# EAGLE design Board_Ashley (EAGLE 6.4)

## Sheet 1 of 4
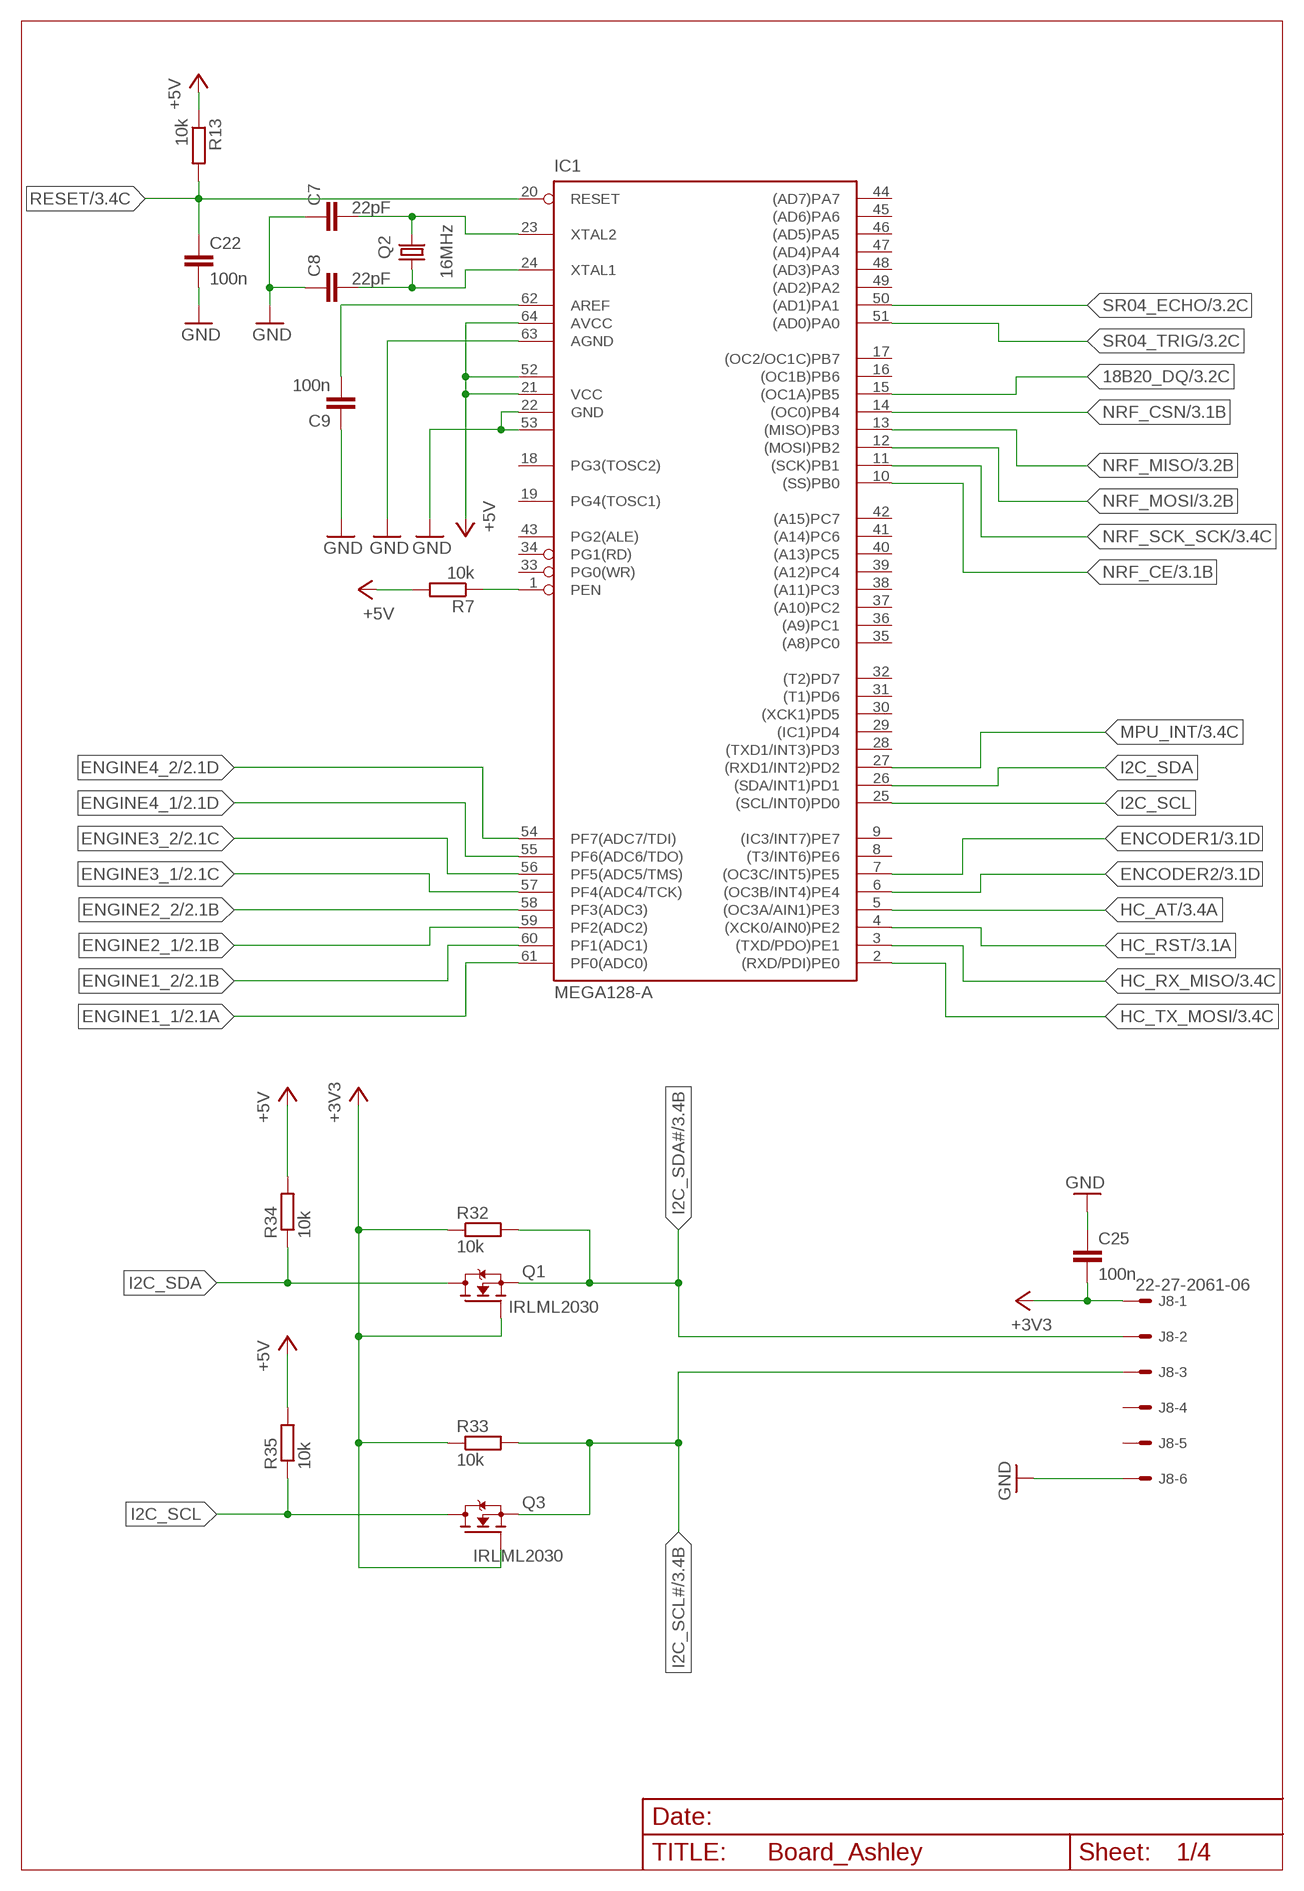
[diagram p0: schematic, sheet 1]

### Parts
C7  22pF  C-EUC0805  [C0805]
C8  22pF  C-EUC0805  [C0805]
C9  100n  C-EUC0805  [C0805]
C22  100n  C-EUC0805  [C0805]
C25  100n  C-EUC0805  [C0805]
IC1  MEGA128-A  [TQFP64]
J8  22-27-2061-06  [6410-06]
Q1  IRLML2030  [SOT23]
Q2  16MHz  CRYSTALHC49U-V  [HC49U-V]
Q3  IRLML2030  [SOT23]
R7  10k  R-EU_R0805  [R0805]
R13  10k  R-EU_R0805  [R0805]
R32  10k  R-EU_R0805  [R0805]
R33  10k  R-EU_R0805  [R0805]
R34  10k  R-EU_R0805  [R0805]
R35  10k  R-EU_R0805  [R0805]

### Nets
18B20_DQ: IC1.15((OC1A)PB5) ; also sheet 3
+3V3: C25.2 J8.1 Q1.1(G) Q3.1(G) R32.1 R33.1 ; also sheet 3,4
+5V: IC1.21(VCC) IC1.52(VCC1) IC1.64(AVCC) R7.2 R13.1 R34.2 R35.2 ; also sheet 3,4
ENCODER1: IC1.7((OC3C/INT5)PE5) ; also sheet 3
ENCODER2: IC1.6((OC3B/INT4)PE4) ; also sheet 3
ENGINE1_1: IC1.61(PF0(ADC0)) ; also sheet 2
ENGINE1_2: IC1.60(PF1(ADC1)) ; also sheet 2
ENGINE2_1: IC1.59(PF2(ADC2)) ; also sheet 2
ENGINE2_2: IC1.58(PF3(ADC3)) ; also sheet 2
ENGINE3_1: IC1.57(PF4(ADC4/TCK)) ; also sheet 2
ENGINE3_2: IC1.56(PF5(ADC5/TMS)) ; also sheet 2
ENGINE4_1: IC1.55(PF6(ADC6/TDO)) ; also sheet 2
ENGINE4_2: IC1.54(PF7(ADC7/TDI)) ; also sheet 2
GND: C7.1 C8.1 C9.1 C22.2 C25.1 IC1.22(GND) IC1.53(GND1) IC1.63(AGND) J8.6 ; also sheet 2,3,4
HC_AT: IC1.5((OC3A/AIN1)PE3) ; also sheet 3
HC_RST: IC1.4((XCK0/AIN0)PE2) ; also sheet 3
HC_RX_MISO: IC1.3((TXD/PDO)PE1) ; also sheet 3
HC_TX_MOSI: IC1.2((RXD/PDI)PE0) ; also sheet 3
I2C_SCL: IC1.25((SCL/INT0)PD0) Q3.3(D) R35.1
I2C_SCL#: J8.3 Q3.2(S) R33.2 ; also sheet 3
I2C_SDA: IC1.26((SDA/INT1)PD1) Q1.3(D) R34.1
I2C_SDA#: J8.2 Q1.2(S) R32.2 ; also sheet 3
MPU_INT: IC1.27((RXD1/INT2)PD2) ; also sheet 3
N$13: C8.2 IC1.24(XTAL1) Q2.1
N$15: C7.2 IC1.23(XTAL2) Q2.2
N$16: C9.2 IC1.62(AREF)
N$17: IC1.1(PEN) R7.1
NRF_CE: IC1.10((SS)PB0) ; also sheet 3
NRF_CSN: IC1.14((OC0)PB4) ; also sheet 3
NRF_MISO: IC1.13((MISO)PB3) ; also sheet 3
NRF_MOSI: IC1.12((MOSI)PB2) ; also sheet 3
NRF_SCK_SCK: IC1.11((SCK)PB1) ; also sheet 3
RESET: C22.1 IC1.20(RESET) R13.2 ; also sheet 3
SR04_ECHO: IC1.50((AD1)PA1) ; also sheet 3
SR04_TRIG: IC1.51((AD0)PA0) ; also sheet 3
Unconnected: IC1.8((T3/INT6)PE6) IC1.9((IC3/INT7)PE7) IC1.16((OC1B)PB6) IC1.17((OC2/OC1C)PB7) IC1.18(PG3(TOSC2)) IC1.19(PG4(TOSC1)) IC1.28((TXD1/INT3)PD3) IC1.29((IC1)PD4) IC1.30((XCK1)PD5) IC1.31((T1)PD6) IC1.32((T2)PD7) IC1.33(PG0(WR)) IC1.34(PG1(RD)) IC1.35((A8)PC0) IC1.36((A9)PC1) IC1.37((A10)PC2) IC1.38((A11)PC3) IC1.39((A12)PC4) IC1.40((A13)PC5) IC1.41((A14)PC6) IC1.42((A15)PC7) IC1.43(PG2(ALE)) IC1.44((AD7)PA7) IC1.45((AD6)PA6) IC1.46((AD5)PA5) IC1.47((AD4)PA4) IC1.48((AD3)PA3) IC1.49((AD2)PA2) J8.4 J8.5

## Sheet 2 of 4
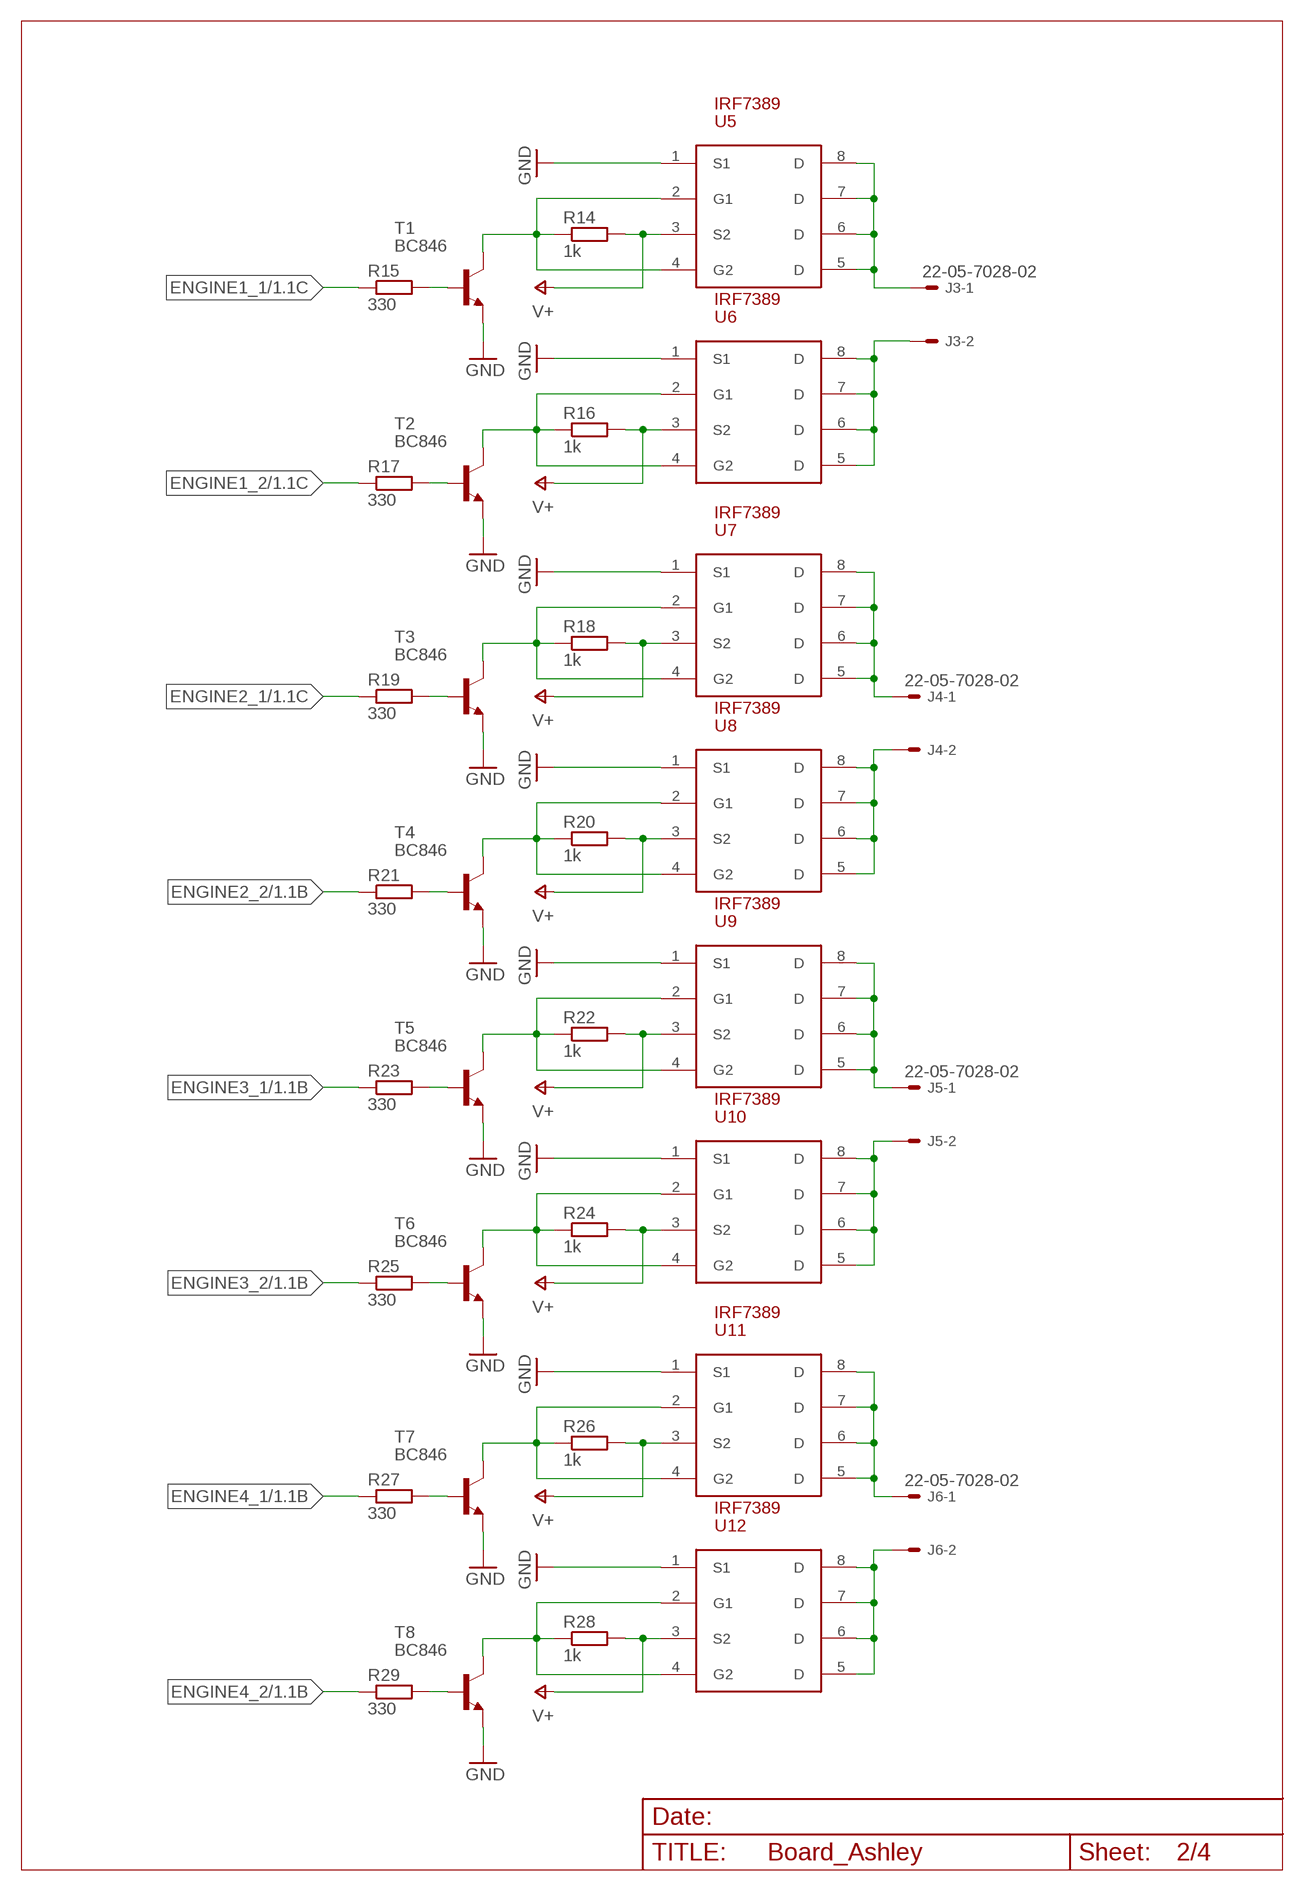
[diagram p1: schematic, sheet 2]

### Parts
J3  22-05-7028-02  [7395-02]
J4  22-05-7028-02  [7395-02]
J5  22-05-7028-02  [7395-02]
J6  22-05-7028-02  [7395-02]
R14  1k  R-EU_R0805  [R0805]
R15  330  R-EU_R0805  [R0805]
R16  1k  R-EU_R0805  [R0805]
R17  330  R-EU_R0805  [R0805]
R18  1k  R-EU_R0805  [R0805]
R19  330  R-EU_R0805  [R0805]
R20  1k  R-EU_R0805  [R0805]
R21  330  R-EU_R0805  [R0805]
R22  1k  R-EU_R0805  [R0805]
R23  330  R-EU_R0805  [R0805]
R24  1k  R-EU_R0805  [R0805]
R25  330  R-EU_R0805  [R0805]
R26  1k  R-EU_R0805  [R0805]
R27  330  R-EU_R0805  [R0805]
R28  1k  R-EU_R0805  [R0805]
R29  330  R-EU_R0805  [R0805]
T1  BC846  [SOT23]
T2  BC846  [SOT23]
T3  BC846  [SOT23]
T4  BC846  [SOT23]
T5  BC846  [SOT23]
T6  BC846  [SOT23]
T7  BC846  [SOT23]
T8  BC846  [SOT23]
U5  IRF7389  [SO-08M]
U6  IRF7389  [SO-08M]
U7  IRF7389  [SO-08M]
U8  IRF7389  [SO-08M]
U9  IRF7389  [SO-08M]
U10  IRF7389  [SO-08M]
U11  IRF7389  [SO-08M]
U12  IRF7389  [SO-08M]

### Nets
ENGINE1_1: R15.1 ; also sheet 1
ENGINE1_2: R17.1 ; also sheet 1
ENGINE2_1: R19.1 ; also sheet 1
ENGINE2_2: R21.1 ; also sheet 1
ENGINE3_1: R23.1 ; also sheet 1
ENGINE3_2: R25.1 ; also sheet 1
ENGINE4_1: R27.1 ; also sheet 1
ENGINE4_2: R29.1 ; also sheet 1
GND: T1.2(E) T2.2(E) T3.2(E) T4.2(E) T5.2(E) T6.2(E) T7.2(E) T8.2(E) U5.1(S1) U6.1(S1) U7.1(S1) U8.1(S1) U9.1(S1) U10.1(S1) U11.1(S1) U12.1(S1) ; also sheet 1,3,4
N$10: J3.1 U5.5(D) U5.6(D) U5.7(D) U5.8(D)
N$27: J3.2 U6.5(D) U6.6(D) U6.7(D) U6.8(D)
N$29: J4.1 U7.5(D) U7.6(D) U7.7(D) U7.8(D)
N$31: R18.1 T3.3(C) U7.2(G1) U7.4(G2)
N$32: R19.2 T3.1(B)
N$34: J4.2 U8.5(D) U8.6(D) U8.7(D) U8.8(D)
N$35: R20.1 T4.3(C) U8.2(G1) U8.4(G2)
N$36: R14.1 T1.3(C) U5.2(G1) U5.4(G2)
N$37: R16.1 T2.3(C) U6.2(G1) U6.4(G2)
N$38: R21.2 T4.1(B)
N$40: J5.1 U9.5(D) U9.6(D) U9.7(D) U9.8(D)
N$41: R22.1 T5.3(C) U9.2(G1) U9.4(G2)
N$42: R23.2 T5.1(B)
N$44: R17.2 T2.1(B)
N$46: J5.2 U10.5(D) U10.6(D) U10.7(D) U10.8(D)
N$47: R15.2 T1.1(B)
N$49: R24.1 T6.3(C) U10.2(G1) U10.4(G2)
N$50: R25.2 T6.1(B)
N$52: J6.1 U11.5(D) U11.6(D) U11.7(D) U11.8(D)
N$53: R26.1 T7.3(C) U11.2(G1) U11.4(G2)
N$54: R27.2 T7.1(B)
N$56: J6.2 U12.5(D) U12.6(D) U12.7(D) U12.8(D)
N$57: R28.1 T8.3(C) U12.2(G1) U12.4(G2)
N$58: R29.2 T8.1(B)
V+: R14.2 R16.2 R18.2 R20.2 R22.2 R24.2 R26.2 R28.2 U5.3(S2) U6.3(S2) U7.3(S2) U8.3(S2) U9.3(S2) U10.3(S2) U11.3(S2) U12.3(S2) ; also sheet 4

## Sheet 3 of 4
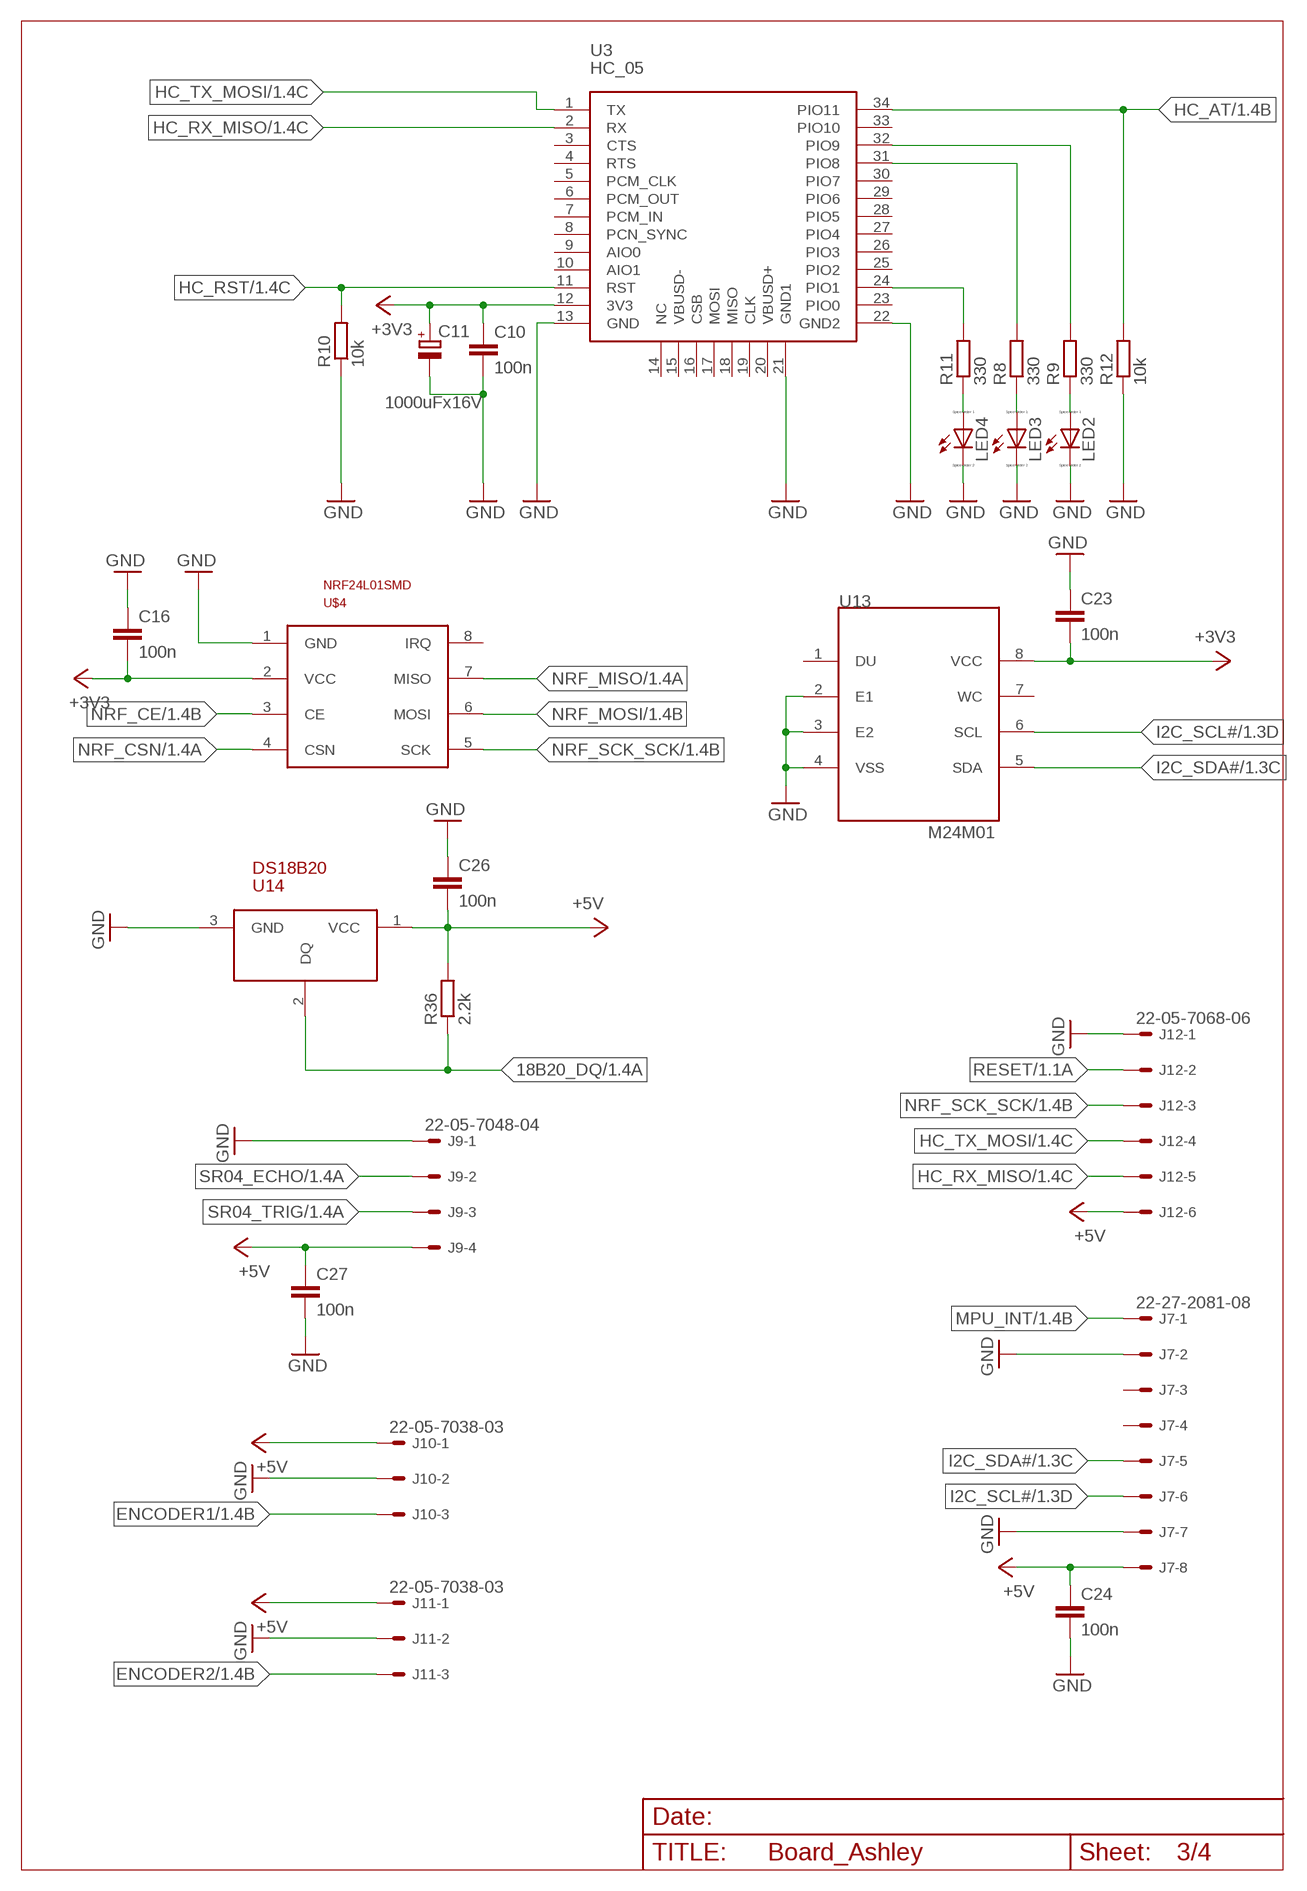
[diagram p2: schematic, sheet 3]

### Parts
C10  100n  C-EUC0805  [C0805]
C11  1000uFx16V  CPOL-EUG  [PANASONIC_G]
C16  100n  C-EUC0805  [C0805]
C23  100n  C-EUC0805  [C0805]
C24  100n  C-EUC0805  [C0805]
C26  100n  C-EUC0805  [C0805]
C27  100n  C-EUC0805  [C0805]
J7  22-27-2081-08  [6410-08]
J9  22-05-7048-04  [7395-04]
J10  22-05-7038-03  [7395-03]
J11  22-05-7038-03  [7395-03]
J12  22-05-7068-06  [7395-06]
LED2  LED_E  [LED_1206]
LED3  LED_E  [LED_1206]
LED4  LED_E  [LED_1206]
R8  330  R-EU_R0805  [R0805]
R9  330  R-EU_R0805  [R0805]
R10  10k  R-EU_R0805  [R0805]
R11  330  R-EU_R0805  [R0805]
R12  10k  R-EU_R0805  [R0805]
R36  2.2k  R-EU_R0805  [R0805]
U3  HC_05  [BLUETOOTH_SMD]
U13  M24M01  [SO-08M]
U14  DS18B20  [TO92-LINE]
U$4  NRF24L01SMD  [NRF24L01SMD]

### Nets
18B20_DQ: R36.1 U14.2(DQ) ; also sheet 1
+3V3: C10.1 C11.+ C16.2 C23.2 U3.12(3V3) U13.8(VCC) U$4.2(VCC) ; also sheet 1,4
+5V: C24.1 C26.2 C27.1 J7.8 J9.4 J10.1 J11.1 J12.6 R36.2 U14.1(VCC) ; also sheet 1,4
ENCODER1: J10.3 ; also sheet 1
ENCODER2: J11.3 ; also sheet 1
GND: C10.2 C11.- C16.1 C23.1 C24.2 C26.1 C27.2 J7.2 J7.7 J9.1 J10.2 J11.2 J12.1 LED2.C LED3.C LED4.C R10.1 R12.1 U3.13(GND) U3.21(GND1) U3.22(GND2) U13.2(E1) U13.3(E2) U13.4(VSS) U14.3(GND) U$4.1(GND) ; also sheet 1,2,4
HC_AT: R12.2 U3.34(PIO11) ; also sheet 1
HC_RST: R10.2 U3.11(RST) ; also sheet 1
HC_RX_MISO: J12.5 U3.2(RX) ; also sheet 1
HC_TX_MOSI: J12.4 U3.1(TX) ; also sheet 1
I2C_SCL#: J7.6 U13.6(SCL) ; also sheet 1
I2C_SDA#: J7.5 U13.5(SDA) ; also sheet 1
MPU_INT: J7.1 ; also sheet 1
N$14: R8.2 U3.31(PIO8)
N$18: R9.2 U3.32(PIO9)
N$19: LED3.A R8.1
N$21: LED2.A R9.1
N$24: R11.2 U3.24(PIO1)
N$25: LED4.A R11.1
NRF_CE: U$4.3(CE) ; also sheet 1
NRF_CSN: U$4.4(CSN) ; also sheet 1
NRF_MISO: U$4.7(MISO) ; also sheet 1
NRF_MOSI: U$4.6(MOSI) ; also sheet 1
NRF_SCK_SCK: J12.3 U$4.5(SCK) ; also sheet 1
RESET: J12.2 ; also sheet 1
SR04_ECHO: J9.2 ; also sheet 1
SR04_TRIG: J9.3 ; also sheet 1
Unconnected: J7.3 J7.4 U3.3(CTS) U3.4(RTS) U3.5(PCM_CLK) U3.6(PCM_OUT) U3.7(PCM_IN) U3.8(PCN_SYNC) U3.9(AIO0) U3.10(AIO1) U3.14(NC) U3.15(VBUSD-) U3.16(CSB) U3.17(MOSI) U3.18(MISO) U3.19(CLK) U3.20(VBUSD+) U3.23(PIO0) U3.25(PIO2) U3.26(PIO3) U3.27(PIO4) U3.28(PIO5) U3.29(PIO6) U3.30(PIO7) U3.33(PIO10) U13.1(DU) U13.7(WC) U$4.8(IRQ)

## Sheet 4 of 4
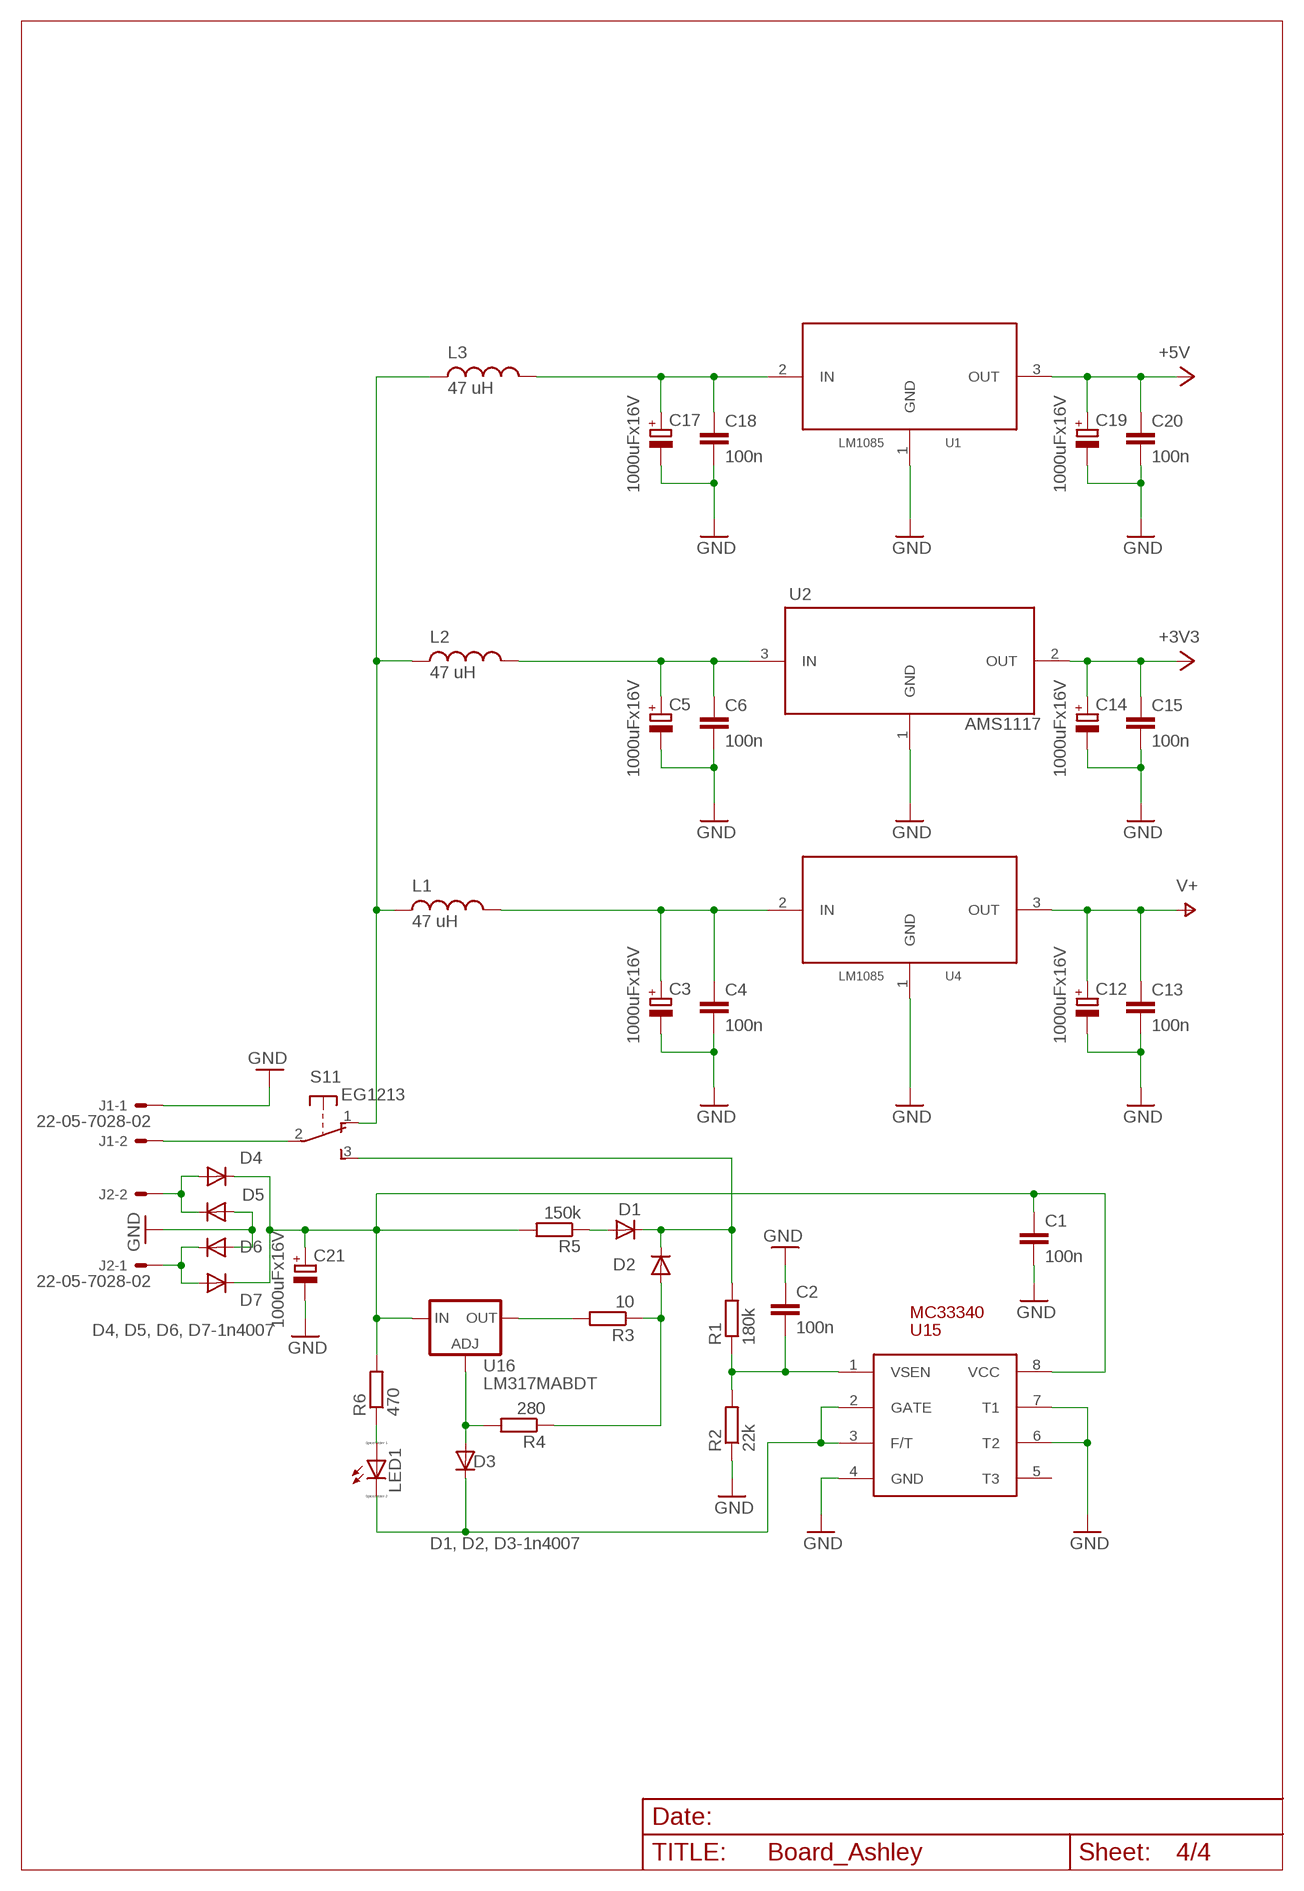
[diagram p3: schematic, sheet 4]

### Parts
C1  100n  C-EUC0805  [C0805]
C2  100n  C-EUC0805  [C0805]
C3  1000uFx16V  CPOL-EUG  [PANASONIC_G]
C4  100n  C-EUC0805  [C0805]
C5  1000uFx16V  CPOL-EUG  [PANASONIC_G]
C6  100n  C-EUC0805  [C0805]
C12  1000uFx16V  CPOL-EUG  [PANASONIC_G]
C13  100n  C-EUC0805  [C0805]
C14  1000uFx16V  CPOL-EUG  [PANASONIC_G]
C15  100n  C-EUC0805  [C0805]
C17  1000uFx16V  CPOL-EUG  [PANASONIC_G]
C18  100n  C-EUC0805  [C0805]
C19  1000uFx16V  CPOL-EUG  [PANASONIC_G]
C20  100n  C-EUC0805  [C0805]
C21  1000uFx16V  CPOL-EUG  [PANASONIC_G]
D1  1N4004  [DO41-10]
D2  1N4004  [DO41-10]
D3  1n4007  1N4004  [DO41-10]
D4  1N4004  [DO41-10]
D5  1N4004  [DO41-10]
D6  1N4004  [DO41-10]
D7  1N4004  [DO41-10]
J1  22-05-7028-02  [7395-02]
J2  22-05-7028-02  [7395-02]
L1  47 uH  MSS1260  [MSS1260]
L2  47 uH  MSS1260  [MSS1260]
L3  47 uH  MSS1260  [MSS1260]
LED1  LED_E  [LED_1206]
R1  180k  R-EU_R0805  [R0805]
R2  22k  R-EU_R0805  [R0805]
R3  10  R-EU_R0805  [R0805]
R4  280  R-EU_R0805  [R0805]
R5  150k  R-EU_R0805  [R0805]
R6  470  R-EU_R0805  [R0805]
S1  EG1213  [EG1213]
U1  LM1085  [TO263]
U2  AMS1117  [SOT223R_INFINEON]
U4  LM1085  [TO263]
U15  MC33340  [SO8]
U16  LM317MABDT  [DPACK]

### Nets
+3V3: C14.+ C15.1 U2.2(OUT) ; also sheet 1,3
+5V: C19.+ C20.1 U1.3(OUT) ; also sheet 1,3
GND: C1.2 C2.1 C3.- C4.2 C5.- C6.2 C12.- C13.2 C14.- C15.2 C17.- C18.2 C19.- C20.2 C21.- D5.A D6.A J1.1 R2.1 U1.1(GND) U2.1(GND) U4.1(GND) U15.4(GND) U15.6(T2) U15.7(T1) ; also sheet 1,2,3
N$1: C5.+ C6.1 L2.P$1 U2.3(IN)
N$2: D3.C LED1.C U15.2(GATE) U15.3(F/T)
N$3: C2.2 R1.1 R2.2 U15.1(VSEN)
N$4: J1.2 S1.2(1:P)
N$5: D2.A R3.1 R4.1
N$6: R3.2 U16.4(OUT)
N$7: D3.A R4.2 U16.1(ADJ)
N$8: D1.C D2.C R1.2 S1.3(1:S)
N$9: D1.A R5.1
N$11: LED1.A R6.1
N$12: C3.+ C4.1 L1.P$1 U4.2(IN)
N$20: L1.P$2 L2.P$2 L3.P$2 S1.1(1:O)
N$22: C17.+ C18.1 L3.P$1 U1.2(IN)
N$26: D4.A D5.C J2.2
N$28: D6.C D7.A J2.1
N$30: C1.1 C21.+ D4.C D7.C R5.2 R6.2 U15.8(VCC) U16.3(IN)
V+: C12.+ C13.1 U4.3(OUT) ; also sheet 2
Unconnected: S1.MT1(MT) S1.MT2(MT) U15.5(T3)

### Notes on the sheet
- D4, D5, D6, D7-1n4007
- D1, D2, D3-1n4007

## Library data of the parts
C1 C2 C4 C6-C10 C13 C15 C16 C18 C20 C22-C27 = rcl:C-EU: CAPACITOR, European symbol
C3 C5 C11 C12 C14 C17 C19 C21 = rcl:CPOL-EU: POLARIZED CAPACITOR, European symbol
D1-D7 = diode:1N4004: DIODE
IC1 = avr-7:MEGA128: MICROCONTROLLER 128 Kbytes FLASH 4 Kbytes SRAM 4 Kbytes EEPROM DUAL USART 8-channel 10 bit ADC
J1-J6 = con-molex:22-?-02: CONNECTOR
J7 = con-molex:22-?-08: CONNECTOR wire to board 2.54 mm (.1 inch) pitch header
J8 J12 = con-molex:22-?-06: CONNECTOR wire to board 2.54 mm (.1 inch) pitch header
J9 = con-molex:22-?-04: CONNECTOR wire to board 2.54 mm (.1 inch) pitch header
J10 J11 = con-molex:22-?-03: CONNECTOR wire to board 2.54 mm (.1 inch) pitch header
L1-L3 = inductor-coilcraft:MSS1260: SMT Power Inductor
LED1-LED4 = eagle-ltspice:LED_E: LED; SPICEMODEL: NONE; SPICEPREFIX: D; SPICETYPE: diode
Q1 Q3 = IRLML2030:IRLML2030
Q2 = ada:CRYSTAL: CRYSTAL; OC_FARNELL: 1666969; OC_NEWARK: unknown
R1-R29 R32-R36 = rcl:R-EU_: RESISTOR, European symbol
S1 = ada:EG1213: E-Switch right-angle slide SPDT Part #EG1213 http://www.ladyada.net/library/eagle
T1-T8 = transistor:BC846: NPN TRANSISTOR
U1 U4 = LM1085:LM1085
U2 = AMS1117:AMS1117
U3 = hc05:HC_05: HC-05 Bluetooth Module
U5-U12 = IRF7389:IRF7389
U13 = M24M01:M24M01
U14 = DS18b20:DS18B20
U15 = MC33340:MC33340
U16 = v-reg:LM317?*: 500 mA Adjustable Output Positive Voltage Regulator Source: http://www.onsemi.co.jp .. LM317M-D.PDF
U$4 = nrf24l01smd:NRF24L01SMD

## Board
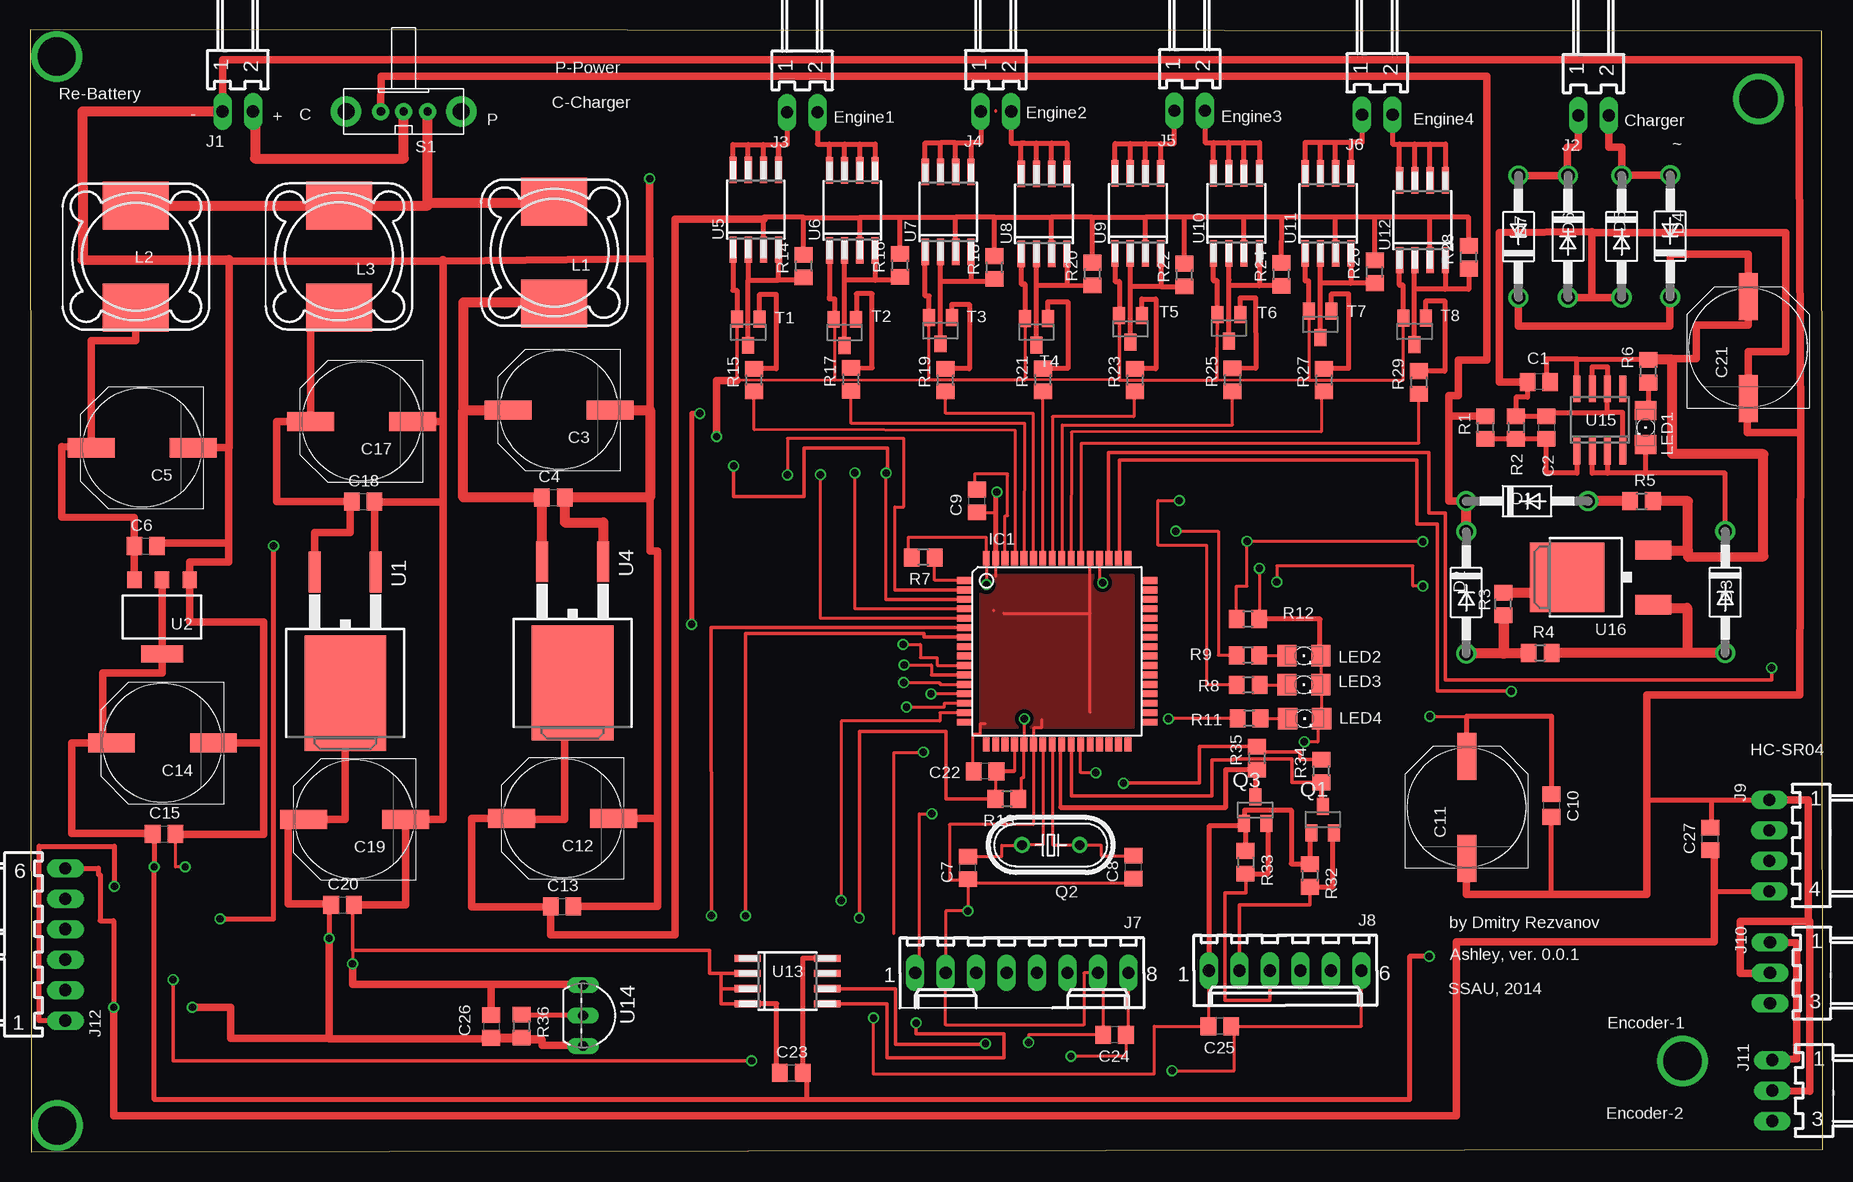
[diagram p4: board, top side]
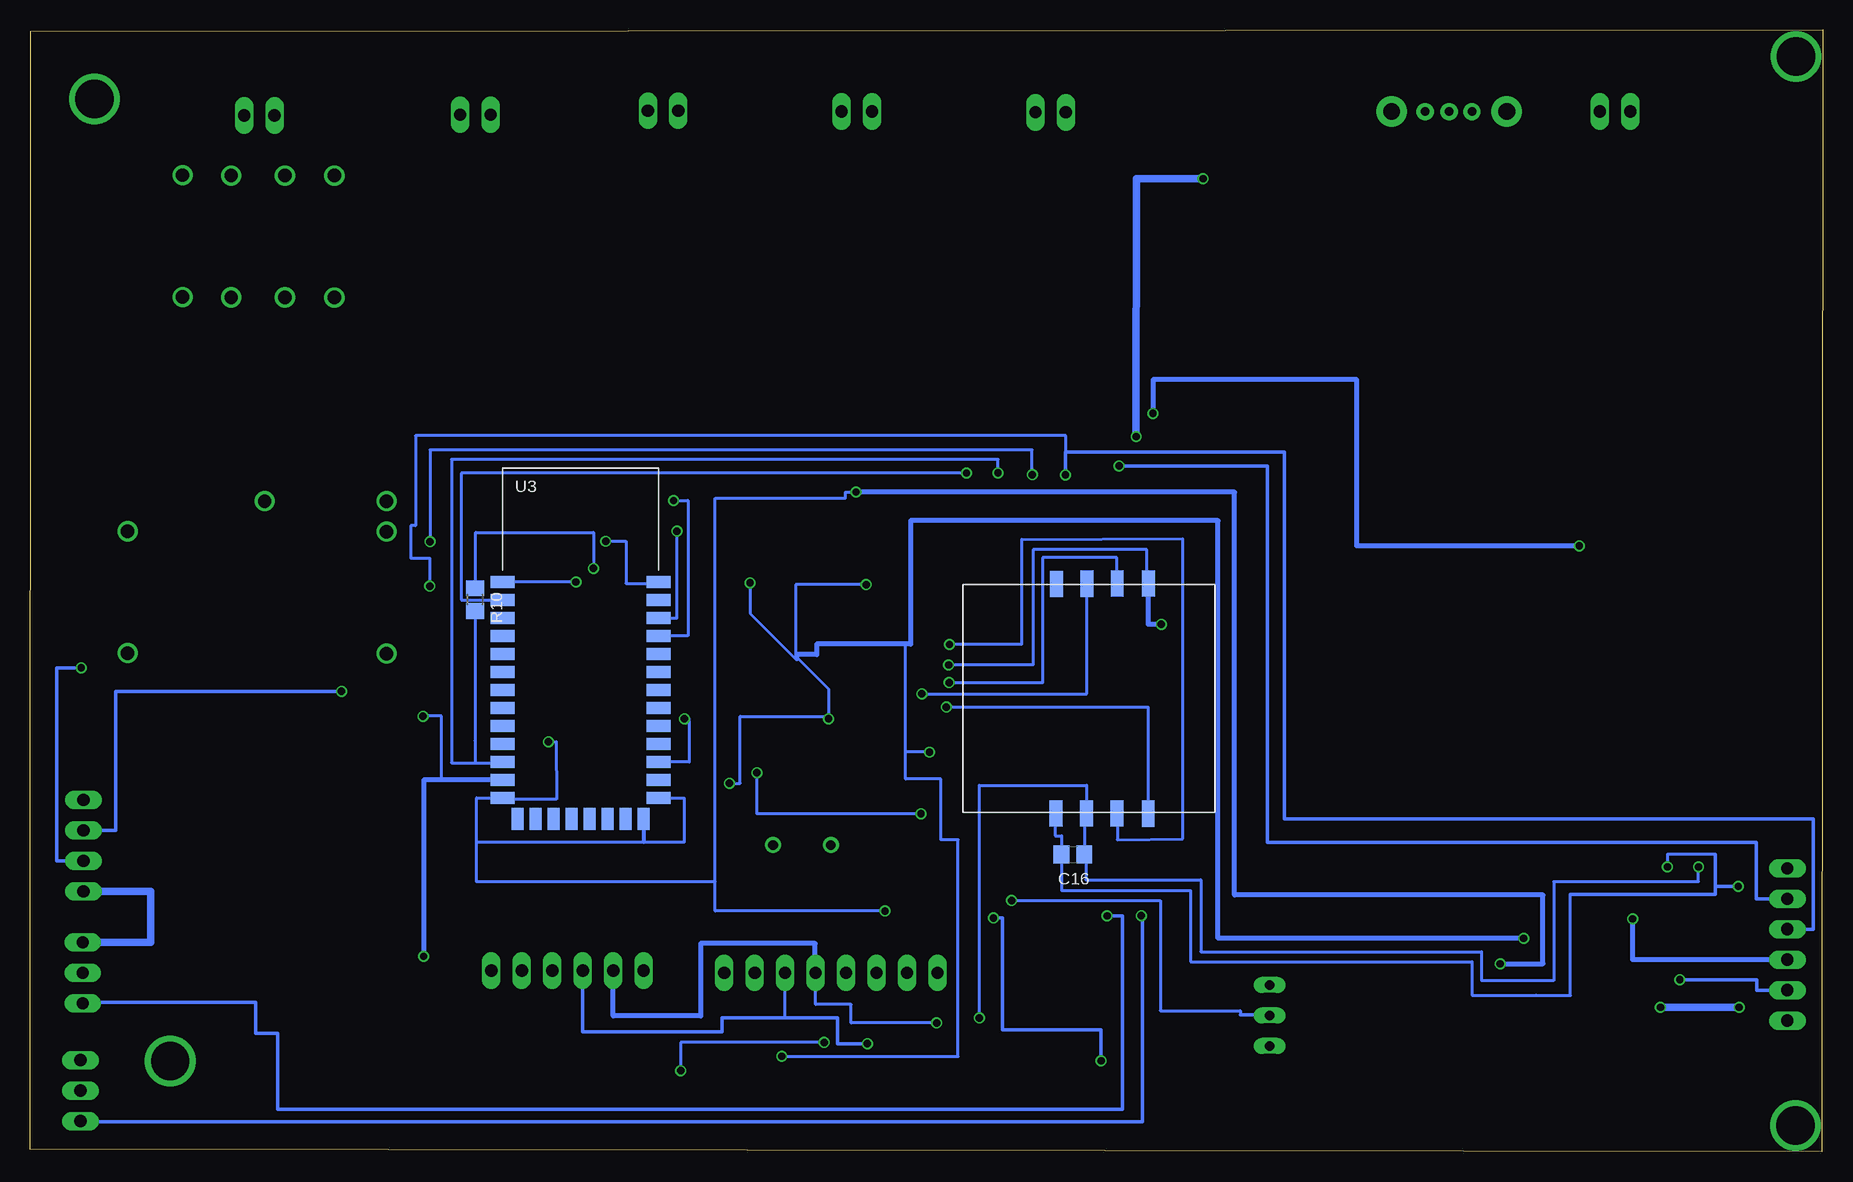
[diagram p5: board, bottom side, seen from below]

Size 149.44 x 93.52 mm. Coordinates in mm from the lower left corner, seen from the top.
Outline: 0.1,0 149.44,0.2 149.37,93.42 0,93.52 0.1,0
Copper layers (1*16): Top 0.035mm / dielectric 1.5mm / Bottom 0.035mm
Design rules "ITEADstudio_DRC": minimum track width 6mil, minimum drill 12mil, track to track 6mil, track to pad 6mil, pad to pad 6mil, via to via 6mil, smd to smd 0mil, copper to edge 10mil, drill to drill 10mil, minimum pad ring 10mil, minimum via ring 6mil, stop-mask expansion 2mil, vias tented up to drill 100mil, thermal gap 10mil

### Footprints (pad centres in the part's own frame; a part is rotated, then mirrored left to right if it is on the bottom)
C0805 = smd 1.3 x 1.5: 1 -0.95,0; 2 0.95,0
PANASONIC_G = smd 3.9 x 1.6: + 4.25,0; - -4.25,0
DO41-10 = drill 1.118: A 5.08,0; C -5.08,0
TQFP64 = smd 1.194 x 0.559: 1 -7.76,5.905; 2 -7.76,5.118; 3 -7.76,4.331; 4 -7.76,3.543; 5 -7.76,2.756; 6 -7.76,1.968; 7 -7.76,1.181; 8 -7.76,0.394; 9 -7.76,-0.394; 10 -7.76,-1.181; 11 -7.76,-1.968; 12 -7.76,-2.756; 13 -7.76,-3.543; 14 -7.76,-4.331; 15 -7.76,-5.118; 16 -7.76,-5.905; 33 7.76,-5.905; 34 7.76,-5.118; 35 7.76,-4.331; 36 7.76,-3.543; 37 7.76,-2.756; 38 7.76,-1.968; 39 7.76,-1.181; 40 7.76,-0.394; 41 7.76,0.394; 42 7.76,1.181; 43 7.76,1.968; 44 7.76,2.756; 45 7.76,3.543; 46 7.76,4.331; 47 7.76,5.118; 48 7.76,5.905 | smd 0.559 x 1.194: 17 -5.905,-7.76; 18 -5.118,-7.76; 19 -4.331,-7.76; 20 -3.543,-7.76; 21 -2.756,-7.76; 22 -1.968,-7.76; 23 -1.181,-7.76; 24 -0.394,-7.76; 25 0.394,-7.76; 26 1.181,-7.76; 27 1.968,-7.76; 28 2.756,-7.76; 29 3.543,-7.76; 30 4.331,-7.76; 31 5.118,-7.76; 32 5.905,-7.76; 49 5.905,7.76; 50 5.118,7.76; 51 4.331,7.76; 52 3.543,7.76; 53 2.756,7.76; 54 1.968,7.76; 55 1.181,7.76; 56 0.394,7.76; 57 -0.394,7.76; 58 -1.181,7.76; 59 -1.968,7.76; 60 -2.756,7.76; 61 -3.543,7.76; 62 -4.331,7.76; 63 -5.118,7.76; 64 -5.905,7.76
7395-02 = drill 1.016 long: 1 1.27,0; 2 -1.27,0
6410-08 = drill 1.016 long: 1 8.89,0; 2 6.35,0; 3 3.81,0; 4 1.27,0; 5 -1.27,0; 6 -3.81,0; 7 -6.35,0; 8 -8.89,0
6410-06 = drill 1.016 long: 1 6.35,0; 2 3.81,0; 3 1.27,0; 4 -1.27,0; 5 -3.81,0; 6 -6.35,0
7395-04 = drill 1.016 long: 1 3.81,0; 2 1.27,0; 3 -1.27,0; 4 -3.81,0
7395-03 = drill 1.016 long: 1 2.54,0; 2 0,0; 3 -2.54,0
7395-06 = drill 1.016 long: 1 6.35,0; 2 3.81,0; 3 1.27,0; 4 -1.27,0; 5 -3.81,0; 6 -6.35,0
MSS1260 = smd 5.5 x 4: P$1 0,4.25; P$2 0,-4.25
LED_1206 = smd 1.6 x 1.803: A -1.422,0; C 1.422,0
SOT23 = smd 1 x 1.4: 1 -0.95,-1.1; 2 0.95,-1.1; 3 0,1.1
HC49U-V = drill 0.813: 1 -2.413,0; 2 2.413,0
R0805 = smd 1.3 x 1.5: 1 -0.95,0; 2 0.95,0
EG1213 = drill 0.7 pad 1.422: 1 -2,0; 2 0,0; 3 1.9,0 | drill 1.4 pad 2.54: MT1 -4.8,0; MT2 4.8,0
TO263 = smd 1 x 3.4: 1 -2.54,-6.6; 2 2.54,-6.6 | smd 6.8 x 9.6: 3 0,3.5
SOT223R_INFINEON = smd 1.2 x 1.4: 1 -2.311,-3.099; 2 0,-3.099; 3 2.311,-3.099 | smd 3.5 x 1.4: 4 0,3.099
BLUETOOTH_SMD = smd 2 x 1: 1 -6.35,3.81; 2 -6.35,2.31; 3 -6.35,0.81; 4 -6.35,-0.69; 5 -6.35,-2.19; 6 -6.35,-3.69; 7 -6.35,-5.19; 8 -6.35,-6.69; 9 -6.35,-8.19; 10 -6.35,-9.69; 11 -6.35,-11.19; 12 -6.35,-12.69; 13 -6.35,-14.19; 22 6.65,-14.19; 23 6.65,-12.69; 24 6.65,-11.19; 25 6.65,-9.69; 26 6.65,-8.19; 27 6.65,-6.69; 28 6.65,-5.19; 29 6.65,-3.69; 30 6.65,-2.19; 31 6.65,-0.69; 32 6.65,0.81; 33 6.65,2.31; 34 6.65,3.81 | smd 1 x 1.8: 14 -5.1,-15.94; 15 -3.6,-15.94; 16 -2.1,-15.94; 17 -0.6,-15.94; 18 0.9,-15.94; 19 2.4,-15.94; 20 3.9,-15.94; 21 5.4,-15.94
SO-08M = smd 0.6 x 2.2: 1 -1.905,-3.33; 2 -0.635,-3.33; 3 0.635,-3.33; 4 1.905,-3.33; 5 1.905,3.33; 6 0.635,3.33; 7 -0.635,3.33; 8 -1.905,3.33
TO92-LINE = drill 0.813 long: 1 2.54,0; 2 0,0; 3 -2.54,0
SO8 = smd 0.6 x 2.2: 1 -1.905,-2.6; 2 -0.635,-2.6; 3 0.635,-2.6; 4 1.905,-2.6; 5 1.905,2.6; 6 0.635,2.6; 7 -0.635,2.6; 8 -1.905,2.6
DPACK = smd 1.6 x 3: 1 -2.28,-4.8; 3 2.28,-4.8 | smd 5.8 x 6.2: 4 0,2.38
NRF24L01SMD = smd 2.184 x 1.067: 1 0,0; 2 0,-2.54; 3 0,-5.08; 4 -0.022,-7.677; 5 19.172,-7.686; 6 19.167,-5.102; 7 19.151,-2.57; 8 19.142,-0.027

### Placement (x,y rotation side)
C1  125.77,64.19 180 top
C2  126.41,60.38 270 top
C3  44.1,61.84 180 top
C4  43.63,54.56 0 top
C5  9.35,58.69 180 top
C6  9.64,50.49 0 top
C7  78.17,23.67 90 top
C8  91.97,23.73 90 top
C9  78.93,54.26 90 top
C10  126.81,28.87 270 top
C11  119.76,28.72 90 top
C12  44.4,27.79 180 top
C13  44.36,20.45 0 top
C14  11.04,34.08 180 top
C15  11.18,26.51 0 top
C16  62.51,24.79 0 bottom
C17  27.64,60.88 180 top
C18  27.77,54.2 0 top
C19  27.06,27.71 180 top
C20  26.06,20.59 0 top
C21  143.23,67.04 90 top
C22  79.62,31.73 180 top
C23  63.46,6.58 0 top
C24  90.4,9.77 180 top
C25  99.18,10.47 180 top
C26  38.45,10.46 270 top
C27  140.07,26.08 90 top
D1  124.8,54.24 0 top
D2  119.72,46.62 270 top
D3  141.31,46.65 270 top
D4  136.72,76.34 90 top
D5  132.67,76.31 270 top
D6  128.19,76.31 270 top
D7  124.07,76.3 90 top
IC1  85.61,41.72 0 top
J1  17.32,86.73 180 top
J2  130.33,86.4 180 top
J3  64.37,86.66 180 top
J4  80.52,86.73 180 top
J5  96.67,86.79 180 top
J6  112.31,86.46 180 top
J7  82.68,14.91 180 top
J8  104.63,15.11 180 top
J9  144.98,25.53 90 top
J10  145.04,14.91 90 top
J11  145.23,5.1 90 top
J12  2.95,17.29 270 top
L1  43.7,74.96 180 top
L2  8.83,74.63 180 top
L3  25.76,74.63 180 top
LED1  134.66,60.38 270 top
LED2  106.18,41.36 0 top
LED3  106.18,38.94 0 top
LED4  106.25,36.12 0 top
Q1  107.76,27.69 0 top
Q2  85.09,25.57 180 top
Q3  102.13,28.48 0 top
R1  121.33,60.38 90 top
R2  123.87,60.38 270 top
R3  122.8,45.67 90 top
R4  125.88,41.6 0 top
R5  134.32,54.24 0 top
R6  134.89,65.07 90 top
R7  74.45,49.56 180 top
R8  101.55,38.91 180 top
R9  101.52,41.39 180 top
R10  112.35,46.04 270 bottom
R11  101.61,36.12 180 top
R12  101.52,44.41 180 top
R13  81.43,29.41 180 top
R14  64.49,73.84 90 top
R15  60.36,64.33 90 top
R16  72.52,73.9 90 top
R17  68.43,64.39 90 top
R18  80.39,73.72 90 top
R19  76.31,64.33 90 top
R20  88.57,73.18 90 top
R21  84.45,64.35 90 top
R22  96.23,73.09 90 top
R23  92.12,64.33 90 top
R24  104.32,73.15 90 top
R25  100.24,64.36 90 top
R26  112.09,73.36 90 top
R27  107.87,64.34 90 top
R28  119.92,74.58 90 top
R29  115.79,64.13 90 top
R32  106.68,23.03 270 top
R33  101.33,24.13 270 top
R34  107.65,31.75 90 top
R35  102.28,32.82 90 top
R36  40.96,10.48 270 top
S1  31.15,86.73 180 top
T1  59.87,68.33 180 top
T2  67.91,68.3 180 top
T3  75.89,68.45 180 top
T4  83.89,68.35 180 top
T5  91.73,68.61 180 top
T6  99.93,68.68 180 top
T7  107.55,68.99 180 top
T8  115.41,68.39 180 top
U1  26.28,41.74 180 top
U2  11,44.59 180 top
U3  103.69,43.69 0 bottom
U4  45.23,42.59 180 top
U5  60.5,78.54 0 top
U6  68.54,78.48 0 top
U7  76.53,78.35 0 top
U8  84.52,78.19 0 top
U9  92.35,78.22 0 top
U10  100.56,78.23 0 top
U11  108.2,78.22 0 top
U12  116.07,77.66 0 top
U13  63.14,14.23 270 top
U14  46.1,11.36 270 top
U15  130.85,61.01 0 top
U16  130.51,47.89 90 top
U$4  63.91,28.2 90 bottom

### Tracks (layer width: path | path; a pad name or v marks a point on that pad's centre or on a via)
18B20_DQ  (via drill 0.61)
  Top 0.254: IC1.15 75.84,36.6 75.85,35.91 67.62,35.9 v67.61,20.94
  Top 0.406: R36.1 46.1,11.43 U14.2
  Bottom 0.152: 46.1,11.42 U14.2
  Bottom 0.254: v67.61,20.94 55.22,20.94 55.22,11.76 48.56,11.76 48.56,11.42
  Bottom 0.305: 48.56,11.42 46.1,11.42
+3V3  (via drill 0.61)
  Top 0.152: 101.33,27.38 101.27,27.38 101.27,27.35
  Top 0.254: U2.2 11.11,47.69 11.11,40 6.1,40 6.1,33.86 3.51,33.86 3.51,26.49 | R33.1 101.33,25.17 | J8.1 98.28,14.47 98.28,10.47 C25.2 98.23,10.46 93.71,10.46 93.71,6.48 70.31,6.48 v70.31,11.16 | v116.68,36.31 119.76,36.31 119.76,36.32 | 66.47,16.12 U13.8
  Top 0.406: 3.51,26.49 10.36,26.49 v10.36,23.75 10.36,4.35 64.72,4.35 | R33.1 101.33,27.38 Q3.1 | 106.7,23.98 R32.1 | C11.+ 119.76,36.32 126.81,36.32 C10.1 | v116.63,16.29 115,16.29 115,4.35 64.72,4.35 | R32.1 106.68,24 105.13,24 105.13,28.48 101.27,28.48 101.27,27.35 101.27,27.17 98.28,27.17 98.28,14.47 | 64.72,4.35 64.72,6.58 C23.2 64.41,16.14 U13.8 | Q1.1 106.68,26.59 R32.1
  Top 0.61: C15.1 10.23,26.54 3.46,26.54 3.46,34.08 6.05,34.08 | 6.05,34.08 C14.+ | U2.2 11,39.93 6.05,39.93 6.05,34.08
  Bottom 0.254: C16.2 61.56,28.2 U$4.2 61.37,30.55 70.31,30.55 v70.31,11.16 | C16.2 61.48,24.79 | C16.2 61.44,24.79 61.44,22.68 51.84,22.68 51.84,16.68 28.44,16.68 28.44,14.26 22.43,14.26 22.43,22.53 10.36,22.53 v10.36,23.75 | U3.12 115.14,31 115.14,36.33 116.68,36.33 v116.68,36.31
  Bottom 0.406: U3.12 116.63,31 v116.63,16.29
+5V  (via drill 0.61)
  Top 0.152: 42.61,9.42 42.61,8.88 42.69,8.88 | U1.3 26.29,36.31
  Top 0.254: IC1.52 89.13,49.48 89.13,47.72 v89.42,47.44 | v82.88,36.1 82.85,36.1 IC1.21 | IC1.64 79.73,49.48 v79.73,47.28 | IC1.21 82.83,33.96 | IC1.64 | R13.1 82.66,29.41 82.66,31.19 82.85,31.19 IC1.21 | C24.1 | J7.8 91.57,9.77 C24.1 | C24.1 91.36,7.95 v86.77,7.95 | v91.14,30.73 | 72.01,18.21 72.01,33.29 74.47,33.29 v74.47,33.31 | IC1.64 79.7,51.24 73.21,51.24 73.21,49.56 R7.2 | 24.94,9.5 24.94,9.66
  Top 0.305: v91.14,30.73 97.47,30.73 97.47,33.78 R35.2 102.28,33.35 105.86,33.35 105.86,32.7 R34.2
  Top 0.406: C20.1 24.94,20.59 v24.94,17.8 | C27.1 140.36,25.13 140.36,21.7 144.98,21.7 J9.4 | J12.6 5.7,23.64 5.7,23.12 5.85,23.12 5.85,19.25 6.98,19.25 v6.98,12.05 | R35.2
  Top 0.61: 21.33,27.71 C19.+ | C19.+ 21.51,27.71 21.51,20.67 25.11,20.67 C20.1 | C27.1 140.38,25.13 140.38,17.48 118.88,17.48 118.88,3 6.98,3 v6.98,12.05 | v13.54,12.05 16.72,12.05 16.72,9.48 24.94,9.48 24.94,9.5 | 41.02,9.44 R36.2 | C26.2 38.45,9.53 R36.2 | v24.94,17.8 24.94,9.66 24.94,9.42 42.61,9.42 | R36.2 40.96,9.34 42.69,9.34 42.69,8.88 46.1,8.88 U14.1 | J10.1 147.29,17.4 147.29,7.74 145.23,7.69 J11.1 | C19.+ 26.29,27.71 26.29,36.31
  Bottom 0.254: v89.42,47.44 89.42,44.9 85.61,41.09 | 85.61,41.09 85.54,41.09 85.39,41.09 82.85,38.55 82.88,38.55 v82.88,36.1 82.88,36.3 90.23,36.3 90.23,30.73 v91.14,30.73 | v79.73,47.28 85.61,47.28 85.61,41.09 | v86.77,7.95 72.07,7.95 72.07,26.01 73.51,26.01 73.51,31.08 76.44,31.08 76.44,33.31 | 76.44,33.31 76.44,42.33 | v74.47,33.31 76.44,33.31
  Bottom 0.406: v24.94,17.8 50.4,17.8 50.4,52.61 76.03,52.61 76.03,42.33 76.44,42.33 83.87,42.33 83.87,41.45 85.54,41.45 85.54,41.09
  Bottom 0.61: v6.98,12.05 v13.54,12.05 | J9.4 139.38,21.72 139.38,17.47 145.56,17.47 145.56,17.45 J10.1
ENCODER1  (via drill 0.61)
  Top 0.305: IC1.7 74.54,42.9 74.54,43.21 59.65,43.21 v59.65,19.67
  Bottom 0.152: 145.04,12.48 J10.3
  Bottom 0.305: v59.65,19.67 58.39,19.67 58.39,3.55 128.79,3.55 128.79,9.87 130.61,9.87 130.61,12.48 145.04,12.48
ENCODER2  (via drill 0.61)
  Top 0.305: IC1.6 56.77,43.71 v56.8,19.69
  Bottom 0.152: v56.8,19.69 56.72,19.69 | 145.23,2.51 J11.3
  Bottom 0.305: 56.72,19.69 56.72,2.51 145.23,2.51
ENGINE1_1
  Top 0.254: IC1.61 82.08,49.48 | IC1.61 | IC1.61 82.13,49.48 82.13,60.13 60.36,60.19 R15.1
ENGINE1_2
  Top 0.254: IC1.60 82.9,49.48 82.92,60.73 68.46,60.73 R17.1
ENGINE2_1
  Top 0.254: 83.68,49.48 IC1.59 | IC1.59 | IC1.59 83.64,61.55 76.31,61.55 R19.1
ENGINE2_2
  Top 0.254: IC1.58 84.45,49.37 R21.1
ENGINE3_1
  Top 0.254: 85.24,49.48 IC1.57 85.21,61.28 92.02,61.28 92.02,63.38 R23.1
ENGINE3_2
  Top 0.254: 85.97,49.48 IC1.56 86.04,49.48 86.04,60.59 100.24,60.59 R25.1
ENGINE4_1
  Top 0.254: R27.1 107.65,63.38 107.65,60.02 86.79,60 IC1.55
ENGINE4_2
  Top 0.254: IC1.54 87.63,49.48 87.63,59.07 115.79,59.09 R29.1
GND  (via drill 0.61)
  Top 0.152: U14.3 45.87,13.9 45.87,13.97 | U1.1 28.72,48.34 28.72,48.47
  Top 0.254: LED3.C 107.64,38.94 | LED3.C 107.7,38.85 107.7,36.12 LED4.C 107.35,36.12 107.35,34.17 106.22,34.17 v106.22,34.19 | LED2.C LED3.C | 88.36,36.64 88.36,44.9 | 88.36,44.9 IC1.53 | 81.16,44.9 88.36,44.9 | 84.34,36.01 84.34,35.37 83.7,35.37 83.7,33.96 IC1.22 83.64,27.28 76.64,27.28 76.64,22.68 78.17,22.68 C7.1 | IC1.63 80.49,48.98 | 80.49,48.98 80.49,47.97 | T4.2 82.93,64.47 82.9,64.33 | 67.08,69.31 67.07,64.39 | 67.07,64.39 67.08,64.32 | 58.92,64.32 T1.2 | 74.92,64.43 74.93,64.34 | 74.93,64.34 T3.2 | 67.07,64.39 74.93,64.34 | 58.92,71.82 58.96,64.33 67.07,64.39 | 82.9,64.33 74.93,64.34 | T5.2 90.75,64.36 82.9,64.33 | 90.79,72.55 90.79,64.32 98.95,64.33 T6.2 | 98.98,72.61 98.96,64.36 106.6,64.34 | 106.6,64.34 110.43,64.33 114.46,64.33 T8.2 | T7.2 106.6,64.34 | 80.35,45.11 80.35,45.15 | 91.7,22.4 78.17,22.4 v78.17,20.07 76.33,20.07 J7.2 76.33,10.56 87.85,10.56 87.85,14.91 J7.7 89.45,14.91 C24.2 83.24,9.77 v83.24,9.11 | 91.7,22.4 92.07,22.4 | 79.61,35.71 79.22,35.71 79.22,34.84 78.6,34.84 78.6,31.73 C22.2 | 80.47,48.98 80.49,48.98 | v12.94,23.75 12.13,23.75 C15.2 | C20.2 26.89,20.59 | 26.89,16.78 v26.89,15.67 | 80.49,53.31 80.49,53.17 | C9.1 80.49,53.31 80.49,53.42 | J8.6 110.98,10.47 C25.1 100.38,10.47 100.38,6.77 v95.2,6.77 | C26.1 | C8.1 91.7,22.78 91.7,22.4 | v102.47,48.64 R12.1
  Top 0.305: 26.89,20.59 26.89,16.78 56.65,16.78 56.65,14.87 57.61,14.87 | U13.2 57.61,14.87 | 57.61,14.87 57.61,13.6 | 57.61,13.6 57.61,12.33 U13.4 | U13.3 57.61,13.6
  Top 0.406: U15.7 130.22,65.46 131.49,65.46 U15.6 131.49,61.65 | U15.4 132.76,61.65 131.49,61.65 | 131.49,61.65 126.41,61.65 C2.1 R2.1 123.87,62.92 124.82,62.92 C1.2 | U5.1 58.6,71.82 58.92,71.82 T1.2 | U6.1 66.63,71.23 66.64,71.23 66.64,71.13 67.08,71.13 67.08,69.31 T2.2 | U8.1 82.62,72.35 82.93,72.35 82.93,69.45 T4.2 | T3.2 74.94,71.34 74.62,71.34 U7.1 | U9.1 90.45,72.55 90.79,72.55 90.79,69.71 T5.2 | T6.2 98.98,72.61 98.66,72.61 U10.1 | T7.2 106.6,72.59 106.3,72.59 U11.1 | T8.2 114.46,72.25 114.15,72.25 114.15,74.33 U12.1 | v80.58,55 80.49,55 80.49,53.42 80.49,53.17 IC1.63 | C11.- 119.72,24.47 | 119.72,21.47 126.81,21.47 C10.2 | LED2.C 107.54,41.36 107.54,44.4 R12.1 | C27.2 140.19,27.03 140.19,29.32 | 140.19,29.32 144.98,29.32 J9.1 | 134.76,29.33 140.19,29.33 140.19,29.32 | J12.1 0.77,10.94 0.77,25.48 7.04,25.48 v7.04,22.13 | C23.1 62.23,6.58 62.23,12.34 59.81,12.34 U13.4
  Top 0.61: 48.33,61.84 C3.- | C17.- 34.42,60.88 | 34.42,60.88 34.42,54.16 | 34.42,54.16 28.72,54.17 | 28.72,48.47 28.72,54.17 | 28.72,54.17 C18.2 | C6.2 10.59,50.75 16.58,50.75 | 16.58,50.75 16.58,49.16 13.32,49.16 U2.1 13.33,47.69 13.33,44.17 19.46,44.17 19.46,34.08 | 16.58,50.75 16.58,58.69 C5.- 16.6,58.69 16.6,74.35 | C15.2 12.13,26.47 19.47,26.47 19.47,34.08 19.46,34.08 | 19.46,34.08 C14.- | C19.- 31.31,27.63 | C19.- 31.31,27.48 | C19.- 31.32,20.59 C20.2 | 34.42,54.16 34.42,27.71 C19.- | 16.6,74.26 34.42,74.26 34.42,60.88 | 34.42,74.27 51.67,74.46 | 51.67,74.46 51.67,61.84 | C13.2 52.3,20.45 52.3,27.81 | 52.3,27.81 48.07,27.81 48.07,27.61 48.65,27.61 C12.- | 51.67,74.46 51.7,74.46 51.7,50.1 52.3,50.1 52.3,27.81 | 51.67,74.46 51.65,74.46 v51.65,81.13 | v57.23,59.63 57.23,64.31 58.92,64.31 58.92,64.32 | D5.A 130.17,71.23 | 130.17,71.23 D6.A | 130.17,76.61 146.36,76.62 146.36,66.7 143.23,66.69 C21.- 143.15,62.79 143.15,59.97 147.59,59.97 | 130.17,76.61 130.17,71.23 | 130.17,76.61 130.17,76.69 122.5,76.63 122.46,64.19 C1.2 | 119.72,24.47 119.72,21.47 134.76,21.47 134.76,29.33 134.76,38.08 147.5,38.08 147.59,59.97 | 147.59,59.97 147.44,91.03 16.05,91.03 J1.1 | v26.89,15.67 26.89,13.97 38.44,13.97 | 45.87,13.97 38.44,13.97 | C26.1 38.44,11.4 38.44,13.97 | J11.2 148.36,5.06 148.36,19.2 148.25,19.22 | 148.25,19.22 142.56,19.22 142.56,14.86 145.04,14.86 J10.2 | 148.25,19.22 148.25,29.35 J9.1
  Top 0.813: C3.- 51.67,61.84 51.67,54.56 C4.2 | C4.2 | C4.2 44.58,52.47 47.77,52.47 U4.1 | 34.42,74.27 34.42,74.26 | J1.1 4.37,86.72 4.38,74.37 16.6,74.35 16.6,74.26
  Bottom 0.152: 8.98,21.46 8.98,21.51 8.98,22.13
  Bottom 0.254: U$4.1 64,28.2 64,26.35 63.46,26.35 | 63.46,26.35 C16.1 63.31,24.79 | v78.17,20.07 92.33,20.07 92.33,22.54 | 92.33,22.54 92.33,54.49 81.48,54.49 81.48,54.99 v80.58,54.99 v80.58,55 | 63.46,26.35 63.44,26.35 63.44,21.78 52.69,21.78 52.69,15.86 29.23,15.86 29.23,13.06 23.88,13.06 21.04,13.04 21.05,21.46 | 8.98,24.81 12.94,24.81 v12.94,23.75 | v83.24,9.11 95.2,9.11 v95.2,6.77 | U3.22 94.91,29.5 94.91,25.8 98.29,25.8 U3.21 98.27,27.75 98.27,25.78 112.23,25.78 112.23,29.5 | 112.23,29.5 U3.13 110.04,29.38 105.56,29.38 105.57,34.19 v106.22,34.19 106.22,34.15 | 112.23,29.5 112.25,29.5 112.25,22.54 92.33,22.54 | R10.1 112.29,46.99 112.29,51.64 102.47,51.64 | 102.47,51.64 | 102.47,51.64 v102.47,48.64
  Bottom 0.305: 21.05,21.46 8.98,21.46 8.98,22.13 | v7.04,22.13 8.98,22.13 | 8.98,24.81 8.98,22.13
  Bottom 0.406: v26.89,15.67 23.32,15.67 23.32,21.42 49.03,21.42 49.03,54.99 v80.58,54.99 v80.58,55
  Bottom 0.61: v51.65,81.13 57.19,81.13 v57.23,59.63
  pour Top (isolate 0.305): 79.26,48.07 91.96,48.07 91.96,35.37 79.26,35.37
HC_AT  (via drill 0.61)
  Top 0.254: 77.85,44.41 IC1.5 65.89,44.48 v65.89,56.44 | v116.1,50.87 101.45,50.87 v101.45,50.9 101.45,47.17 100.55,47.17 100.55,44.41 R12.2
  Bottom 0.254: v65.89,56.44 65.92,56.44 65.92,58.52 116.1,58.52 v116.1,50.87 | v101.45,50.9 99.76,50.9 99.76,47.38 97.04,47.38 U3.34
HC_RST  (via drill 0.61)
  Top 0.254: 77.83,45.24 IC1.4 68.75,45.27 v68.75,56.6
  Bottom 0.254: v68.75,56.6 68.75,57.73 114.31,57.73 114.31,32.43 112.34,32.43 | 112.34,32.43 110.04,32.43 U3.11 | R10.2 112.34,34.27 112.34,32.43
HC_RX_MISO  (via drill 0.61)
  Top 0.152: 71.37,46.05 71.4,46.05 71.4,56.53
  Top 0.254: 71.37,46.05 v71.37,56.58
  Top 0.305: IC1.3 71.37,46.05 | 71.4,56.53 71.46,56.53 71.46,58.65 64.5,58.65 64.5,54.62 58.66,54.62 v58.66,57.18
  Bottom 0.254: v71.37,56.58 113.49,56.58 113.49,46.02 110.04,46.02 U3.2
  Bottom 0.305: v58.66,57.18 46.28,57.18 46.28,25.8 5.55,25.8 5.55,21.1 J12.5
HC_TX_MOSI  (via drill 0.61)
  Top 0.254: IC1.2 77.85,46.88 | 72.09,46.84 72.09,53.76 72.84,53.76 72.84,59.46 63.13,59.46 v63.13,56.43 | v116.11,47.15 115.27,47.15 115.27,48.84 103.93,48.84 v103.93,47.5
  Top 0.305: 72.09,46.84 IC1.2
  Bottom 0.254: v63.13,56.43 63.1,56.43 63.1,59.02 63.1,59.03 63.1,59.71 117.31,59.69 117.31,52.21 117.7,52.21 117.7,49.5 116.11,49.5 v116.11,47.15 | v103.93,47.5 U3.1
  Bottom 0.305: J12.4 0.79,18.56 0.79,27.77 44.87,27.77 44.87,58.32 63.13,58.32 v63.13,56.43
I2C_SCL
  Top 0.254: IC1.25 85.9,33.96
  Top 0.305: 85.9,33.96 85.9,28.73
  Top 0.406: 85.9,28.73 99.69,28.73 99.69,31.87 R35.1 102.13,31.87 Q3.3
I2C_SCL#  (via drill 0.61)
  Top 0.152: Q3.2 103.23,27.38 103.23,27.36
  Top 0.254: 79.64,8.97 v79.64,9.01
  Top 0.305: 79.64,8.97 72.15,8.97 72.15,13.6 U13.6 | 103.23,23.18 101.35,23.18 101.35,21.58 99.6,21.58 99.6,12.64 103.36,12.64 J8.3
  Top 0.406: R33.2 103.23,23.18 103.23,27.36
  Bottom 0.254: 86.49,11.18 J7.6
  Bottom 0.305: v79.64,9.01 82.13,9.01 82.13,11.18 86.49,11.18 91.73,11.18 91.73,10.01 103.36,10.01 J8.3
I2C_SDA
  Top 0.152: Q1.3 107.65,28.79 107.65,28.39
  Top 0.254: IC1.26
  Top 0.305: IC1.26 86.8,29.69 98.51,29.69 98.51,32.65 100.31,32.65 100.31,32.77 105.2,32.77 105.2,30.81 107.65,30.81 R34.1
  Top 0.406: R34.1 107.65,28.39
I2C_SDA#  (via drill 0.61)
  Top 0.152: Q1.2 108.62,26.59 108.62,26.19
  Top 0.254: J8.2
  Top 0.305: v73.86,10.74 73.85,9.85 81.19,9.85 81.19,7.85 71.44,7.85 71.44,12.33 U13.5 | J8.2 100.81,15.11 100.81,20.58 106.68,20.58 R32.2
  Top 0.406: R32.2 108.62,22.09 108.62,26.19
  Bottom 0.254: v73.86,10.74 80.99,10.74 80.99,12.27 83.95,12.27 J7.5
  Bottom 0.406: J7.5 83.99,14.91 83.99,17.36 93.54,17.36 93.54,11.32 100.82,11.32 J8.2
MPU_INT  (via drill 0.61)
  Top 0.254: 87.6,33.96 IC1.27 87.58,31.6 v88.85,31.6 | J7.1 74.14,14.91 74.14,28.17 v75.17,28.17 v75.17,28.19
  Bottom 0.254: v75.17,28.19 88.85,28.19 v88.85,31.6
N$1
  Top 0.61: C5.+ 5.1,58.74 | 5.1,58.74 2.64,58.8 2.64,52.93 8.7,52.88 8.7,51 | 8.7,51 C6.1 | U2.3 8.69,51 8.7,51 | 5.1,58.74 5.1,67.61 8.83,67.61 L2.P$1
N$2
  Top 0.406: U15.3 131.49,56.57 | 131.49,56.57 130.22,56.57 U15.2 | LED1.C 134.66,56.57 | 134.66,56.57 131.49,56.57 | D3.C 141.31,56.57 134.66,56.57
N$3
  Top 0.406: U15.1 128.95,56.57 126.41,56.57 C2.2 R2.2 R1.1
N$4
  Top 0.813: J1.2 18.75,86.45 18.75,82.81 31.15,82.81 S1.2
N$5
  Top 0.813: R4.1 124.93,41.54 122.89,41.54 122.89,44.72 R3.1 122.8,41.54 D2.A
N$6
  Top 0.813: R3.2 122.99,46.62 125.43,46.62 125.43,47.89 U16.4
N$7
  Top 0.813: U16.1 135.31,45.35 138.13,45.35 138.13,41.6 | 138.13,41.6 R4.2 | D3.A 141.31,41.6 138.13,41.6
N$8
  Top 0.61: 29.13,86.73 S1.3 29.26,89.68 121.45,89.68 121.44,66 119.06,66 119.06,63.04 118.26,63.04 118.26,61.33 | D1.C 118.26,54.24 118.26,60.89 118.26,61.33 | R1.2 118.26,61.33
  Top 0.813: D2.C D1.C
N$9
  Top 0.813: R5.1 D1.A
N$10
  Top 0.406: U5.8 58.6,83.97 59.87,83.97 | 59.87,83.97 61.14,83.97 | 61.14,83.97 62.41,83.97 U5.5 62.41,83.97 63.13,83.99 63.13,86.7 J3.1 | U5.7 59.87,83.97 | U5.6 61.14,83.97
N$11
  Top 0.406: R6.1 134.89,61.8 LED1.A
N$12
  Top 0.152: U4.2 42.68,49.19 42.68,49.93
  Top 0.813: 36.14,61.84 C3.+ | 42.68,49.42 42.68,49.93 C4.1 36.12,54.56 36.12,61.84 36.14,61.84 | 36.14,61.84 36.14,70.82 43.7,70.82 L1.P$1
N$13
  Top 0.254: IC1.24 85.24,33.96 85.24,25.57 | 85.24,25.57 Q2.1 | 85.24,25.57 89.28,25.57 89.28,24.69 C8.2
N$14  (via drill 0.61)
  Top 0.254: 100.6,38.69 R8.2 98.1,38.91 98.1,50.55 94.02,50.55 94.02,54.3 v95.8,54.3
  Bottom 0.254: v95.8,54.3 94.61,54.3 94.61,43 U3.31
N$15
  Top 0.254: IC1.23 84.43,25.57 Q2.2 82.68,25.56 81.01,25.56 81.01,24.62 C7.2
N$16
  Top 0.254: IC1.62 81.25,49.48 | IC1.62 | IC1.62 81.28,53.04 81.49,53.04 81.49,56.37 81.49,56.52 81.49,56.53 78.77,56.53 78.77,55.21 C9.2
N$17
  Top 0.254: 77.85,47.64 IC1.1 75.4,47.63 R7.1
N$18  (via drill 0.61)
  Top 0.254: 100.57,41.41 R9.2 100.57,41.4 99.04,41.4 99.04,51.74 v95.51,51.74
  Bottom 0.254: U3.32 95.51,44.5 v95.51,51.74
N$19
  Top 0.254: R8.1 104.76,38.91 LED3.A
N$20
  Top 0.61: L3.P$2 L2.P$2 | 44.51,79.07 44.51,78.78 43.7,78.78 L1.P$2
  Top 0.813: L2.P$2 33.15,78.88 33.15,79.07 | 33.15,79.07 S1.1 | 44.51,79.07 33.15,79.07
N$21
  Top 0.254: R9.1 104.76,41.39 LED2.A
N$22
  Top 0.61: L3.P$1 23.39,69.06 C17.+ 20.55,60.88 20.55,54.2 C18.1 26.7,54.2 26.7,51.63 23.75,51.63 23.75,48.13 U1.2
N$24  (via drill 0.61)
  Top 0.254: R11.2 95.25,36.12 v94.89,36.1
  Bottom 0.254: v94.89,36.1 94.48,36.09 94.48,32.5 U3.24
N$25
  Top 0.254: R11.1 LED4.A
N$26
  Top 0.61: 132.67,81.42 D5.C 132.69,81.39 | 132.67,81.42 D4.A | 132.67,81.42 132.67,83.75 131.6,83.75 J2.2
N$27
  Top 0.406: U6.8 66.63,84.02 | 66.63,84.02 67.9,84.02 | 67.9,84.02 69.17,84.02 | 69.17,84.02 70.45,84.02 U6.5 | U6.7 67.9,84.02 | U6.6 69.17,84.02 | J3.2 65.64,84.02 66.63,84.02
N$28
  Top 0.61: D6.C 128.31,81.37 D7.A | 128.25,81.39 D6.C | J2.1 129.06,83.76 128.17,83.76 128.17,81.39 D6.C
N$29
  Top 0.406: U7.8 74.62,84.12 75.89,84.12 | 77.16,84.12 78.43,84.12 | 78.43,84.12 U7.5 | U7.6 77.16,84.12 | 77.16,84.12 75.89,84.12 | U7.7 75.89,84.12 | J4.1 79.25,84.12 78.43,84.12
N$30
  Top 0.406: U15.8 128.95,66.09 | 128.95,66.09 126.41,66.09 | 126.41,66.09 126.41,64.19 C1.1 | 126.41,66.12 126.41,66.09 | 128.95,66.09 135.3,66.09 135.3,66.02 R6.2
  Top 0.61: D7.C 124.07,68.84 136.71,68.84 136.71,71.26 D4.C 136.72,74.83 143.22,74.83 C21.+ | 136.89,66.02 136.89,66.11 138.9,66.11 138.9,68.91 143.22,68.91 C21.+ | C21.+
  Top 0.813: U16.3 135.31,50.14 138.2,50.14 | 138.2,50.14 138.2,54.24 R5.2 | 138.2,50.14 138.2,49.6 144.49,49.63 144.49,58.16 136.89,58.18 136.89,66.02 R6.2
N$31
  Top 0.406: T3.3 75.89,72.56 | 75.89,72.56 U7.2 | U7.4 78.43,72.56 | 78.43,72.56 75.89,72.56 | R18.1 80.39,72.56 78.43,72.56
N$32
  Top 0.406: T3.1 76.84,70.67 78.3,70.67 78.3,65.29 R19.2
N$33  (via drill 3.2 pad 2.54)
  other vias: 2.23,91.32
N$34
  Top 0.406: U8.8 82.62,84.11 | 82.62,84.11 83.89,84.11 | 83.89,84.11 85.16,84.11 | 85.16,84.11 86.43,84.11 U8.5 | U8.6 85.16,84.11 | U8.7 83.89,84.11 | 82.88,84.1 82.62,84.11 | J4.2 81.79,84.11 82.62,84.11
N$35
  Top 0.406: T4.3 83.89,72.22 | 83.89,72.22 U8.2 | U8.4 86.43,72.24 | 83.89,72.22 86.43,72.22 86.43,72.24 | 86.43,72.24 R20.1
N$36
  Top 0.406: U5.2 59.87,72.68 | 59.87,72.68 62.41,72.68 | 62.41,72.68 U5.4 | T1.3 59.87,72.68 | R14.1 64.49,72.68 62.41,72.68
N$37
  Top 0.406: T2.3 67.91,72.65 | 67.91,72.65 U6.2 | U6.4 70.44,72.65 | 70.44,72.65 67.91,72.65 | R16.1 72.52,72.65 70.44,72.65
N$38
  Top 0.406: T4.1 84.84,70.88 86.52,70.88 86.52,65.3 R21.2
N$39  (via drill 3.2 pad 2.54)
  other vias: 144.07,87.76
N$40
  Top 0.406: U9.8 90.45,84.05 91.72,84.05 | 91.72,84.05 92.99,84.05 | 92.99,84.05 94.24,84.05 U9.5 94.26,84.05 95.38,84.05 95.38,86.79 J5.1 | U9.6 92.99,84.05 | U9.7 91.72,84.05
N$41
  Top 0.406: T5.3 91.73,72.14 | 91.73,72.14 91.73,74.89 U9.2 | 91.73,72.14 94.26,72.14 U9.4 94.26,72.14 R22.1
N$42
  Top 0.406: T5.1 92.68,71.09 93.84,71.09 93.84,65.28 R23.2
N$43  (via drill 3.2 pad 2.54)
  other vias: 2.27,2.18
N$44
  Top 0.406: R17.2 68.02,65.35 70.2,65.36 70.2,71.53 68.89,71.53 68.89,69.4 T2.1
N$45  (via drill 3.2 pad 2.54)
  other vias: 137.75,7.57
N$46
  Top 0.406: U10.8 98.66,84.14 | 98.66,84.14 99.93,84.14 | 99.93,84.14 101.2,84.14 | 101.2,84.14 102.48,84.14 102.48,81.56 U10.5 | U10.7 99.93,84.14 | U10.6 101.2,84.14 | J5.2 97.94,84.14 98.66,84.14
N$47
  Top 0.406: T1.1 60.82,71.49 62.2,71.49 62.2,65.28 R15.2
N$49
  Top 0.406: U10.4 102.47,72.19 | 102.47,72.19 99.95,72.19 99.95,72.7 | 99.95,72.7 99.95,74.9 U10.2 | T6.3 99.93,72.7 99.95,72.7 | R24.1 104.72,72.19 102.47,72.19
N$50
  Top 0.406: T6.1 100.88,71.21 102.16,71.21 102.17,65.32 R25.2
N$52
  Top 0.406: U11.8 106.29,84.17 107.56,84.17 | 107.56,84.17 108.83,84.17 | 108.83,84.17 110.1,84.17 | 110.1,84.17 U11.5 | U11.7 107.56,84.17 | U11.6 108.83,84.17 | J6.1 111.04,84.17 110.1,84.17
N$53
  Top 0.406: T7.3 107.55,72.42 | 107.55,72.42 107.55,74.89 U11.2 | U11.4 110.1,72.42 | 110.1,72.42 107.55,72.42 | R26.1 110.1,72.42
N$54
  Top 0.406: T7.1 108.5,71.53 109.9,71.53 109.9,65.3 R27.2
N$56
  Top 0.406: U12.8 114.16,84.01 | 114.16,84.01 115.43,84.01 | 115.43,84.01 116.7,84.01 | 116.7,84.01 117.98,84.01 U12.5 | U12.7 115.43,84.01 | U12.6 116.7,84.01 | J6.2 113.58,84.01 114.16,84.01
N$57
  Top 0.406: T8.3 115.41,71.92 | 115.41,71.92 115.41,74.33 U12.2 | R28.1 119.92,71.92 117.97,71.92 | 117.97,71.92 115.41,71.92 | U12.4 117.97,71.92
N$58
  Top 0.406: T8.1 116.36,70.94 117.94,70.94 117.94,65.08 R29.2
N$68
  Top 0.254: 80.52,86.74 80.52,86.8
NRF_CE  (via drill 0.61)
  Top 0.254: 77.85,40.57 IC1.10 75.62,40.54 75.62,41.2 74.22,41.2 74.22,42.3 v72.79,42.3
  Bottom 0.254: U$4.3 58.79,28.2 58.79,26.02 53.36,26.09 53.36,51.12 66.79,51.04 66.79,42.3 v72.79,42.3
NRF_CSN  (via drill 0.61)
  Top 0.254: IC1.14 76.2,37.39 76.2,37.06 73.06,37.06 v73.06,37.07
  Bottom 0.254: v73.06,37.07 56.23,37.07 U$4.4
NRF_MISO  (via drill 0.61)
  Top 0.254: IC1.13 v75.1,38.18 v75.1,38.19
  Bottom 0.254: v75.1,38.19 61.34,38.19 U$4.7
NRF_MOSI  (via drill 0.61)
  Top 0.254: v72.82,39.12 75.85,39.12 75.85,38.96 IC1.12
  Bottom 0.254: U$4.6 58.85,47.37 58.85,49.54 65.04,49.54 65.04,39.1 72.82,39.1 v72.82,39.12
NRF_SCK_SCK  (via drill 0.61)
  Top 0.254: v72.86,40.59 75.14,40.59 75.14,39.75
  Top 0.305: 75.14,39.75 IC1.11
  Top 0.406: v15.85,19.41 20.3,19.41 v20.3,50.51 | v55.83,61.56 55.15,61.56 v55.15,43.97
  Bottom 0.254: U$4.5 56.35,47.38 56.35,50.2 65.82,50.2 65.82,40.6 72.86,40.6 v72.86,40.59
  Bottom 0.406: J12.3 15.85,16.02 v15.85,19.41 | v20.3,50.51 38.86,50.51 38.86,64.37 55.83,64.37 v55.83,61.56 | v55.15,43.97 56.22,43.97 U$4.5
RESET  (via drill 0.61)
  Top 0.254: IC1.20 82.06,31.74 | 82.06,31.74 82.06,31.73 C22.1 | 82.06,31.74 80.48,31.74 R13.2
  Top 0.305: R13.2 76.34,29.41 76.34,35.04 69.13,35.04 v69.13,19.49 | v60.16,7.59 11.92,7.59 v11.92,14.35
  Bottom 0.305: v69.13,19.49 68.39,19.49 68.39,10.16 66.11,10.16 60.16,10.16 v60.16,7.59 | v11.92,14.35 5.49,14.35 5.49,13.46 2.95,13.46 J12.2
SR04_ECHO  (via drill 0.61)
  Top 0.152: IC1.50 90.8,49.48 | 123.48,38.42 v123.48,38.39
  Top 0.305: 90.8,49.48 90.8,57.67 115.6,57.67 115.6,52.32 117.33,52.32 117.33,38.42 123.48,38.42
  Bottom 0.152: J9.2
  Bottom 0.305: v123.48,38.39 142.27,38.39 142.27,26.79 J9.2
SR04_TRIG  (via drill 0.61)
  Top 0.152: IC1.51 89.91,49.48 | 118.01,53.23 117.99,53.23
  Top 0.305: 89.91,49.48 89.91,58.31 116.61,58.31 116.62,53.23 117.99,53.23 117.99,39.33 145.17,39.33 v145.17,40.34
  Bottom 0.152: J9.3
  Bottom 0.305: v145.17,40.34 147.19,40.34 147.19,24.26 J9.3
V+
  Top 0.254: U5.3 61.19,75.21 61.19,77.77
  Top 0.406: U5.3 61.14,77.91 64.49,77.91 64.49,77.9 | R14.2 64.49,77.9 | U6.3 69.17,77.9 | R16.2 72.52,77.9 69.17,77.9 | U7.3 77.16,77.91 | U8.3 85.16,77.92 | 77.16,77.91 80.39,77.91 R18.2 80.39,77.92 85.16,77.92 | R20.2 88.56,77.9 | 88.56,77.9 85.16,77.92 | R16.2 72.52,77.83 | 64.49,77.9 69.17,77.9 | R16.2 72.52,77.91 77.16,77.91 | U9.3 92.99,77.9 | R22.2 96.23,77.9 | 96.23,77.9 92.99,77.9 | U10.3 101.2,77.9 | 101.2,77.9 96.23,77.9 | R24.2 104.34,77.9 | 104.34,77.9 101.2,77.9 | 88.56,77.9 92.99,77.9 | U11.3 108.83,77.9 | 108.83,77.9 104.34,77.9 | R26.2 112.09,77.9 | 112.09,77.9 108.83,77.9 | U12.3 116.7,77.9 | 116.7,77.9 112.09,77.9 | R28.2 119.92,77.9 116.7,77.9
  Top 0.61: 61.19,77.77 53.77,77.77 53.77,18.07 43.41,18.07 C13.1 43.41,20.44 36.8,20.44 36.8,27.79 C12.+ 40.15,27.71 44.55,27.71 44.55,39.09 U4.3

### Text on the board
tNames: P-Power | Re-Battery | C-Charger | - | + | C | P | Engine1 | Engine2 | Engine3 | Engine4 | Charger | ~ | HC-SR04 | by Dmitry Rezvanov | Ashley, ver. 0.0.1 | SSAU, 2014 | Encoder-1 | Encoder-2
